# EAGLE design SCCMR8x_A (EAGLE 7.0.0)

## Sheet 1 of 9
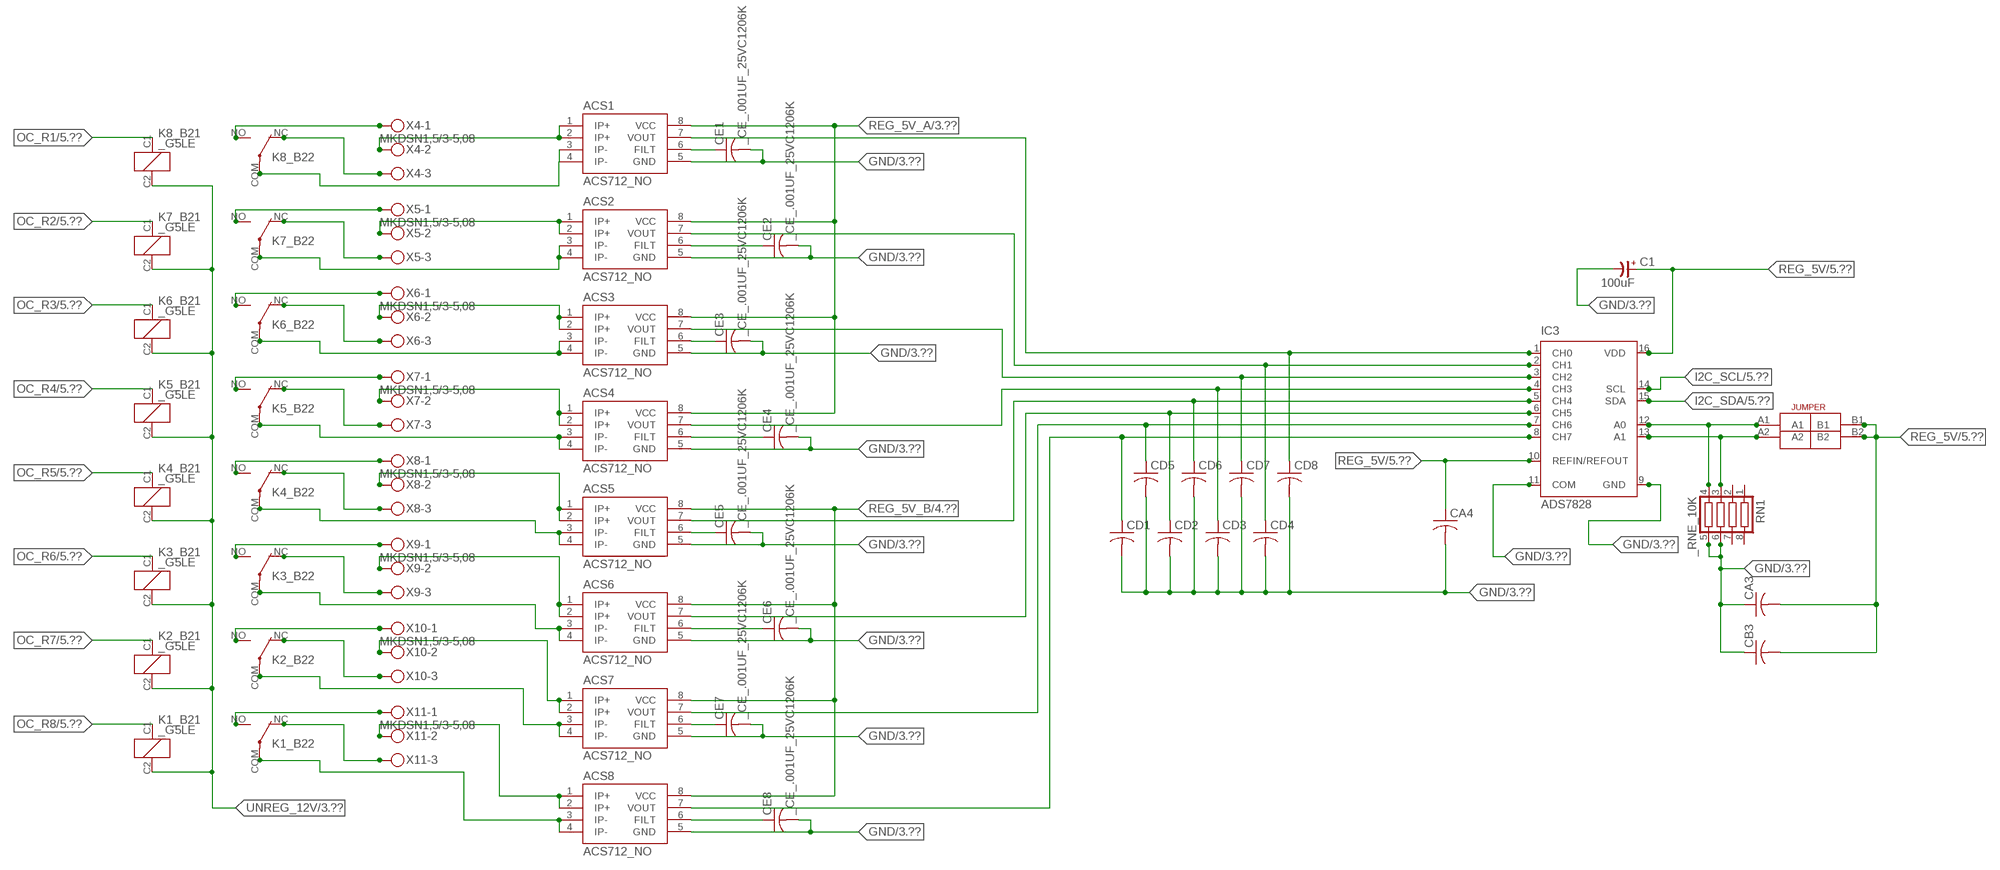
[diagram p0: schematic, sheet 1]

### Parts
ACS1  ACS712_NO  [_MA_DUAL_N-FET]
ACS2  ACS712_NO  [_MA_DUAL_N-FET]
ACS3  ACS712_NO  [_MA_DUAL_N-FET]
ACS4  ACS712_NO  [_MA_DUAL_N-FET]
ACS5  ACS712_NO  [_MA_DUAL_N-FET]
ACS6  ACS712_NO  [_MA_DUAL_N-FET]
ACS7  ACS712_NO  [_MA_DUAL_N-FET]
ACS8  ACS712_NO  [_MA_DUAL_N-FET]
C1  100uF  CP-E-025X060  [E-025X060]
CA3  CC1206KRX7R9BB104C1206K  [CC1206KRX7R9BB104]
CA4  CC1206KRX7R9BB104C1206K  [CC1206KRX7R9BB104]
CB3  TMK316F106ZL-TC1206K  [TMK316F106ZL-T]
CD1  _CD_10NF_50VC1206K  [_CD_10NF_50V]
CD2  _CD_10NF_50VC1206K  [_CD_10NF_50V]
CD3  _CD_10NF_50VC1206K  [_CD_10NF_50V]
CD4  _CD_10NF_50VC1206K  [_CD_10NF_50V]
CD5  _CD_10NF_50VC1206K  [_CD_10NF_50V]
CD6  _CD_10NF_50VC1206K  [_CD_10NF_50V]
CD7  _CD_10NF_50VC1206K  [_CD_10NF_50V]
CD8  _CD_10NF_50VC1206K  [_CD_10NF_50V]
CE1  _CE_.001UF_25VC1206K  [CE]
CE2  _CE_.001UF_25VC1206K  [CE]
CE3  _CE_.001UF_25VC1206K  [CE]
CE4  _CE_.001UF_25VC1206K  [CE]
CE5  _CE_.001UF_25VC1206K  [CE]
CE6  _CE_.001UF_25VC1206K  [CE]
CE7  _CE_.001UF_25VC1206K  [CE]
CE8  _CE_.001UF_25VC1206K  [CE]
IC3  ADS7828  [TSSOP16-PW]
K1_B2  _G5LE  [G5LE]
K2_B2  _G5LE  [G5LE]
K3_B2  _G5LE  [G5LE]
K4_B2  _G5LE  [G5LE]
K5_B2  _G5LE  [G5LE]
K6_B2  _G5LE  [G5LE]
K7_B2  _G5LE  [G5LE]
K8_B2  _G5LE  [G5LE]
RN1  _RNE_10K  [RNE]
U$4  JUMPER_2X2  [JUMPER_2X2]
X4  MKDSN1,5/3-5,08  [MKDSN1,5/3-5,08]
X5  MKDSN1,5/3-5,08  [MKDSN1,5/3-5,08]
X6  MKDSN1,5/3-5,08  [MKDSN1,5/3-5,08]
X7  MKDSN1,5/3-5,08  [MKDSN1,5/3-5,08]
X8  MKDSN1,5/3-5,08  [MKDSN1,5/3-5,08]
X9  MKDSN1,5/3-5,08  [MKDSN1,5/3-5,08]
X10  MKDSN1,5/3-5,08  [MKDSN1,5/3-5,08]
X11  MKDSN1,5/3-5,08  [MKDSN1,5/3-5,08]

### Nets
GND: ACS1.5(GND) ACS2.5(GND) ACS3.5(GND) ACS4.5(GND) ACS5.5(GND) ACS6.5(GND) ACS7.5(GND) ACS8.5(GND) C1.- CA3.1 CA4.2 CB3.1 CD1.2 CD2.2 CD3.2 CD4.2 CD5.2 CD6.2 CD7.2 CD8.2 CE1.2 CE2.2 CE3.2 CE4.2 CE5.2 CE6.2 CE7.2 CE8.2 IC3.9(GND) IC3.11(COM) RN1.5 RN1.6 ; also sheet 3,4,5,7,9
I2C_SCL: IC3.14(SCL) ; also sheet 5,7
I2C_SDA: IC3.15(SDA) ; also sheet 5,7
N$6: ACS5.7(VOUT) CD6.1 IC3.5(CH4)
N$7: ACS1.1(IP+) ACS1.2(IP+) X4.2
N$9: ACS1.7(VOUT) CD8.1 IC3.1(CH0)
N$10: ACS2.7(VOUT) CD4.1 IC3.2(CH1)
N$11: ACS3.7(VOUT) CD7.1 IC3.3(CH2)
N$12: ACS4.7(VOUT) CD3.1 IC3.4(CH3)
N$13: ACS2.1(IP+) ACS2.2(IP+) X5.2
N$14: ACS6.7(VOUT) CD2.1 IC3.6(CH5)
N$15: ACS7.7(VOUT) CD5.1 IC3.7(CH6)
N$17: IC3.12(A0) RN1.4 U$4.A1
N$18: IC3.13(A1) RN1.3 U$4.A2
N$21: ACS4.1(IP+) ACS4.2(IP+) X7.2
N$22: ACS4.3(IP-) ACS4.4(IP-) K5_B2.COM(2:COM)
N$23: ACS5.1(IP+) ACS5.2(IP+) X8.2
N$24: ACS7.1(IP+) ACS7.2(IP+) X10.2
N$25: ACS6.1(IP+) ACS6.2(IP+) X9.2
N$29: ACS8.1(IP+) ACS8.2(IP+) X11.2
N$33: ACS1.6(FILT) CE1.1
N$34: ACS2.6(FILT) CE2.1
N$35: ACS3.6(FILT) CE3.1
N$36: ACS4.6(FILT) CE4.1
N$37: ACS8.7(VOUT) CD1.1 IC3.8(CH7)
N$38: ACS5.6(FILT) CE5.1
N$39: ACS6.6(FILT) CE6.1
N$40: ACS7.6(FILT) CE7.1
N$41: ACS8.6(FILT) CE8.1
N$42: ACS1.3(IP-) ACS1.4(IP-) K8_B2.COM(2:COM)
N$43: K8_B2.NC(2:NC) X4.3
N$44: K8_B2.NO(2:NO) X4.1
N$45: K7_B2.NO(2:NO) X5.1
N$46: K6_B2.NO(2:NO) X6.1
N$137: K7_B2.NC(2:NC) X5.3
N$138: ACS2.3(IP-) ACS2.4(IP-) K7_B2.COM(2:COM)
N$139: K6_B2.NC(2:NC) X6.3
N$140: ACS3.3(IP-) ACS3.4(IP-) K6_B2.COM(2:COM)
N$141: K5_B2.NC(2:NC) X7.3
N$143: K5_B2.NO(2:NO) X7.1
N$144: K4_B2.NO(2:NO) X8.1
N$145: K4_B2.NC(2:NC) X8.3
N$146: ACS5.3(IP-) ACS5.4(IP-) K4_B2.COM(2:COM)
N$147: K3_B2.NO(2:NO) X9.1
N$148: K3_B2.NC(2:NC) X9.3
N$149: ACS6.3(IP-) ACS6.4(IP-) K3_B2.COM(2:COM)
N$150: K2_B2.NO(2:NO) X10.1
N$151: K2_B2.NC(2:NC) X10.3
N$152: ACS7.3(IP-) ACS7.4(IP-) K2_B2.COM(2:COM)
N$153: K1_B2.NO(2:NO) X11.1
N$154: K1_B2.NC(2:NC) X11.3
N$155: ACS8.3(IP-) ACS8.4(IP-) K1_B2.COM(2:COM)
N$166: ACS3.1(IP+) ACS3.2(IP+) X6.2
OC_R1: K8_B2.C1(1:C1) ; also sheet 5
OC_R2: K7_B2.C1(1:C1) ; also sheet 5
OC_R3: K6_B2.C1(1:C1) ; also sheet 5
OC_R4: K5_B2.C1(1:C1) ; also sheet 5
OC_R5: K4_B2.C1(1:C1) ; also sheet 5
OC_R6: K3_B2.C1(1:C1) ; also sheet 5
OC_R7: K2_B2.C1(1:C1) ; also sheet 5
OC_R8: K1_B2.C1(1:C1) ; also sheet 5
REG_5V: C1.+ CA3.2 CA4.1 CB3.2 IC3.10(REFIN/REFOUT) IC3.16(VDD) U$4.B1 U$4.B2 ; also sheet 5,7,9
REG_5V_A: ACS1.8(VCC) ACS2.8(VCC) ACS3.8(VCC) ACS4.8(VCC) ; also sheet 3
REG_5V_B: ACS5.8(VCC) ACS6.8(VCC) ACS7.8(VCC) ACS8.8(VCC) ; also sheet 4
UNREG_12V: K1_B2.C2(1:C2) K2_B2.C2(1:C2) K3_B2.C2(1:C2) K4_B2.C2(1:C2) K5_B2.C2(1:C2) K6_B2.C2(1:C2) K7_B2.C2(1:C2) K8_B2.C2(1:C2) ; also sheet 3,4,5,7
Unconnected: RN1.1 RN1.2 RN1.7 RN1.8

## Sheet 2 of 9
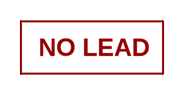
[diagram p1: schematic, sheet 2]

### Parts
U$16  NOPB_LOGO_SYM  [NOPB_LOGO_SYM]

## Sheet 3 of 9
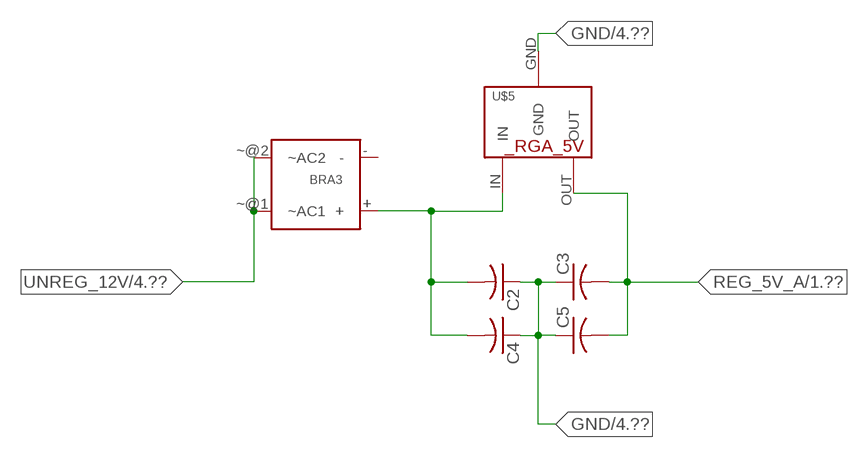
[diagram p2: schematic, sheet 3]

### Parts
BRA3  MB2S_  [MB2S]
C2  _CA_.10UF_50VC1206K  [_CA_.1UF_50V]
C3  _CA_.10UF_50VC1206K  [_CA_.1UF_50V]
C4  _CB_10UF_25VC1206K  [_CB_10UF_25V]
C5  _CB_10UF_25VC1206K  [_CB_10UF_25V]
U$5  _RGA_5V  [_RGA_5V]

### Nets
GND: C2.1 C3.1 C4.1 C5.1 U$5.GND ; also sheet 1,4,5,7,9
N$31: BRA3.+ C2.2 C4.2 U$5.IN
REG_5V_A: C3.2 C5.2 U$5.OUT ; also sheet 1
UNREG_12V: BRA3.~@1(~AC1) BRA3.~@2(~AC2) ; also sheet 1,4,5,7
Unconnected: BRA3.-

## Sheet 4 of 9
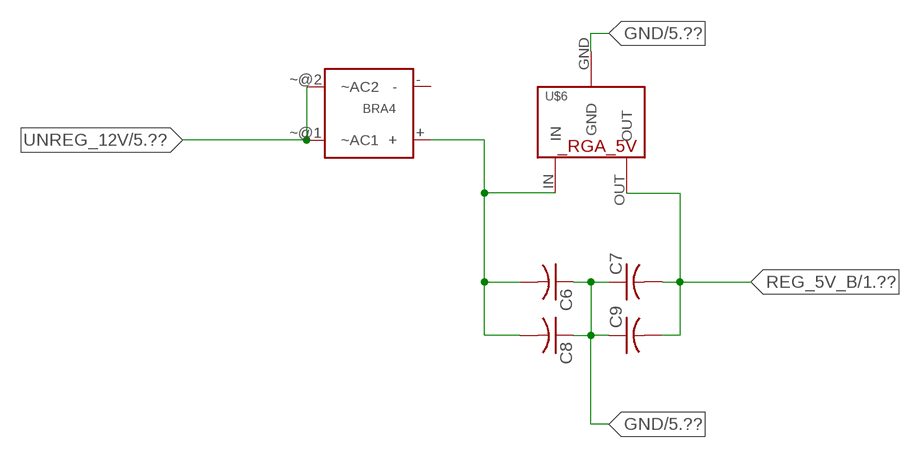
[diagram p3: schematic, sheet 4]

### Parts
BRA4  MB2S_  [MB2S]
C6  _CA_.10UF_50VC1206K  [_CA_.1UF_50V]
C7  _CA_.10UF_50VC1206K  [_CA_.1UF_50V]
C8  _CB_10UF_25VC1206K  [_CB_10UF_25V]
C9  _CB_10UF_25VC1206K  [_CB_10UF_25V]
U$6  _RGA_5V  [_RGA_5V]

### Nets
GND: C6.1 C7.1 C8.1 C9.1 U$6.GND ; also sheet 1,3,5,7,9
N$32: BRA4.+ C6.2 C8.2 U$6.IN
REG_5V_B: C7.2 C9.2 U$6.OUT ; also sheet 1
UNREG_12V: BRA4.~@1(~AC1) BRA4.~@2(~AC2) ; also sheet 1,3,5,7
Unconnected: BRA4.-

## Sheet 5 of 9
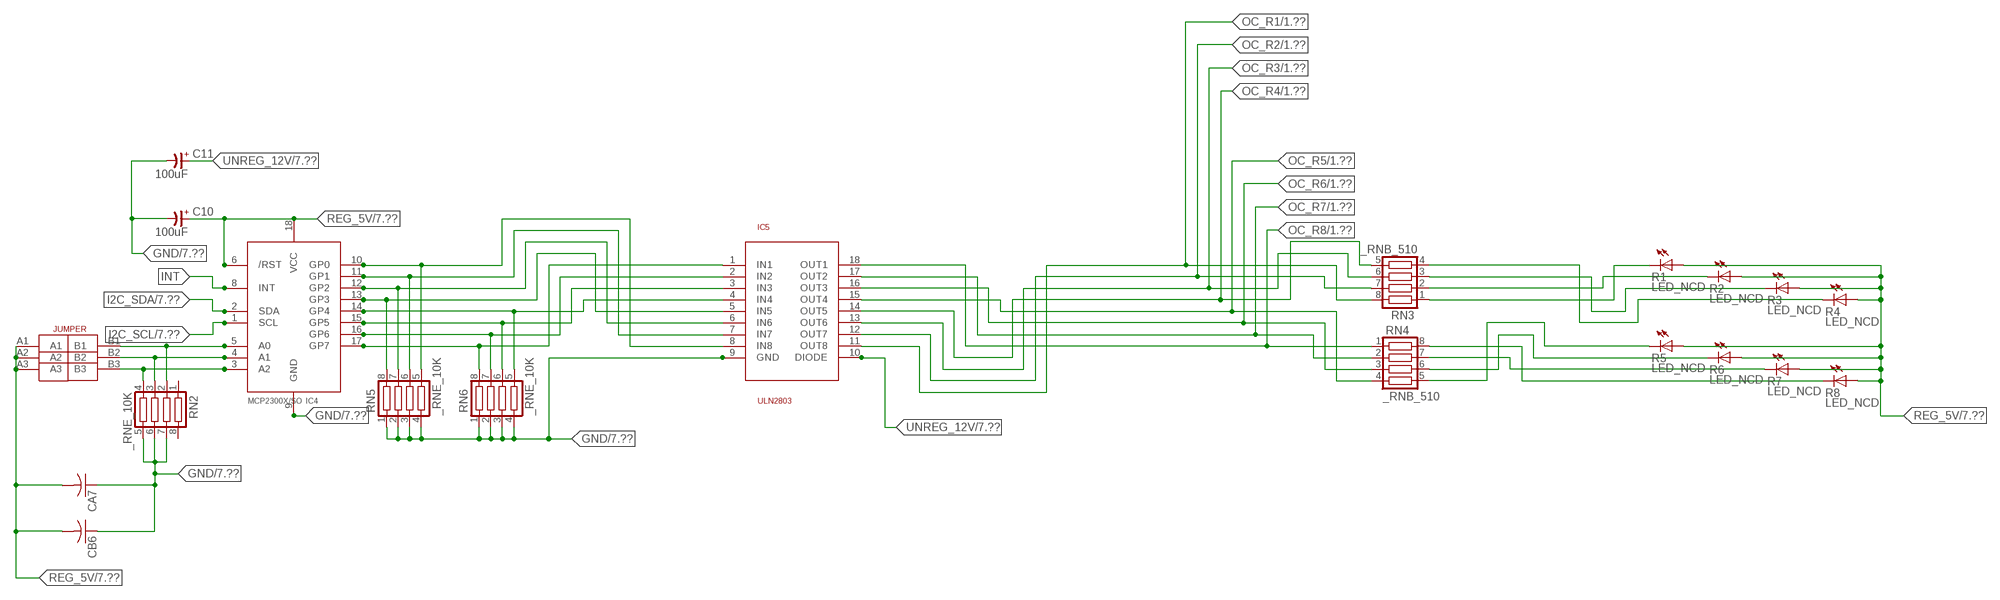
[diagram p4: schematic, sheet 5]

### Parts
C10  100uF  CP-E-025X060  [E-025X060]
C11  100uF  CP-E-025X060  [E-025X060]
CA7  CC1206KRX7R9BB104C1206K  [CC1206KRX7R9BB104]
CB6  TMK316F106ZL-TC1206K  [TMK316F106ZL-T]
IC4  MCP2300X/SO  [SO18W]
IC5  ULN2803  [SO18L]
R1  LED_NCD  [CHIPLED_0603]
R2  LED_NCD  [CHIPLED_0603]
R3  LED_NCD  [CHIPLED_0603]
R4  LED_NCD  [CHIPLED_0603]
R5  LED_NCD  [CHIPLED_0603]
R6  LED_NCD  [CHIPLED_0603]
R7  LED_NCD  [CHIPLED_0603]
R8  LED_NCD  [CHIPLED_0603]
RN2  _RNE_10K  [RNE]
RN3  _RNB_510  [RNB]
RN4  _RNB_510  [RNB]
RN5  _RNE_10K  [RNE]
RN6  _RNE_10K  [RNE]
U$18  JUMPER_3X2  [JUMPER_3X2]

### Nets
GND: C10.- C11.- CA7.1 CB6.1 IC4.9(GND) IC5.9(GND) RN2.5 RN2.6 RN2.7 RN5.1 RN5.2 RN5.3 RN5.4 RN6.1 RN6.2 RN6.3 RN6.4 ; also sheet 1,3,4,7,9
GP4: IC4.14(GP4) IC5.4(IN4) RN6.5
GP6: IC4.16(GP6) IC5.2(IN2) RN6.7
I2C_SCL: IC4.1(SCL) ; also sheet 1,7
I2C_SDA: IC4.2(SDA) ; also sheet 1,7
INT: IC4.8(INT)
N$47: IC4.5(A0) RN2.2 U$18.B1
N$48: IC4.4(A1) RN2.3 U$18.B2
N$49: IC4.3(A2) RN2.4 U$18.B3
N$50: IC4.12(GP2) IC5.6(IN6) RN5.7
N$51: IC4.11(GP1) IC5.7(IN7) RN5.6
N$52: IC4.10(GP0) IC5.8(IN8) RN5.5
N$53: R1.C RN3.1
N$54: R2.C RN3.2
N$55: R3.C RN3.3
N$56: R4.C RN3.4
N$57: R8.C RN4.8
N$81: R7.C RN4.7
N$82: R6.C RN4.6
N$83: R5.C RN4.5
N$89: IC4.13(GP3) IC5.5(IN5) RN5.8
N$93: IC4.15(GP5) IC5.3(IN3) RN6.6
N$94: IC4.17(GP7) IC5.1(IN1) RN6.8
OC_R1: IC5.11(OUT8) RN3.8 ; also sheet 1
OC_R2: IC5.12(OUT7) RN3.7 ; also sheet 1
OC_R3: IC5.13(OUT6) RN3.6 ; also sheet 1
OC_R4: IC5.14(OUT5) RN3.5 ; also sheet 1
OC_R5: IC5.15(OUT4) RN4.4 ; also sheet 1
OC_R6: IC5.16(OUT3) RN4.3 ; also sheet 1
OC_R7: IC5.17(OUT2) RN4.2 ; also sheet 1
OC_R8: IC5.18(OUT1) RN4.1 ; also sheet 1
REG_5V: C10.+ CA7.2 CB6.2 IC4.6(/RST) IC4.18(VCC) R1.A R2.A R3.A R4.A R5.A R6.A R7.A R8.A U$18.A1 U$18.A2 U$18.A3 ; also sheet 1,7,9
UNREG_12V: C11.+ IC5.10(DIODE) ; also sheet 1,3,4,7
Unconnected: RN2.1 RN2.8

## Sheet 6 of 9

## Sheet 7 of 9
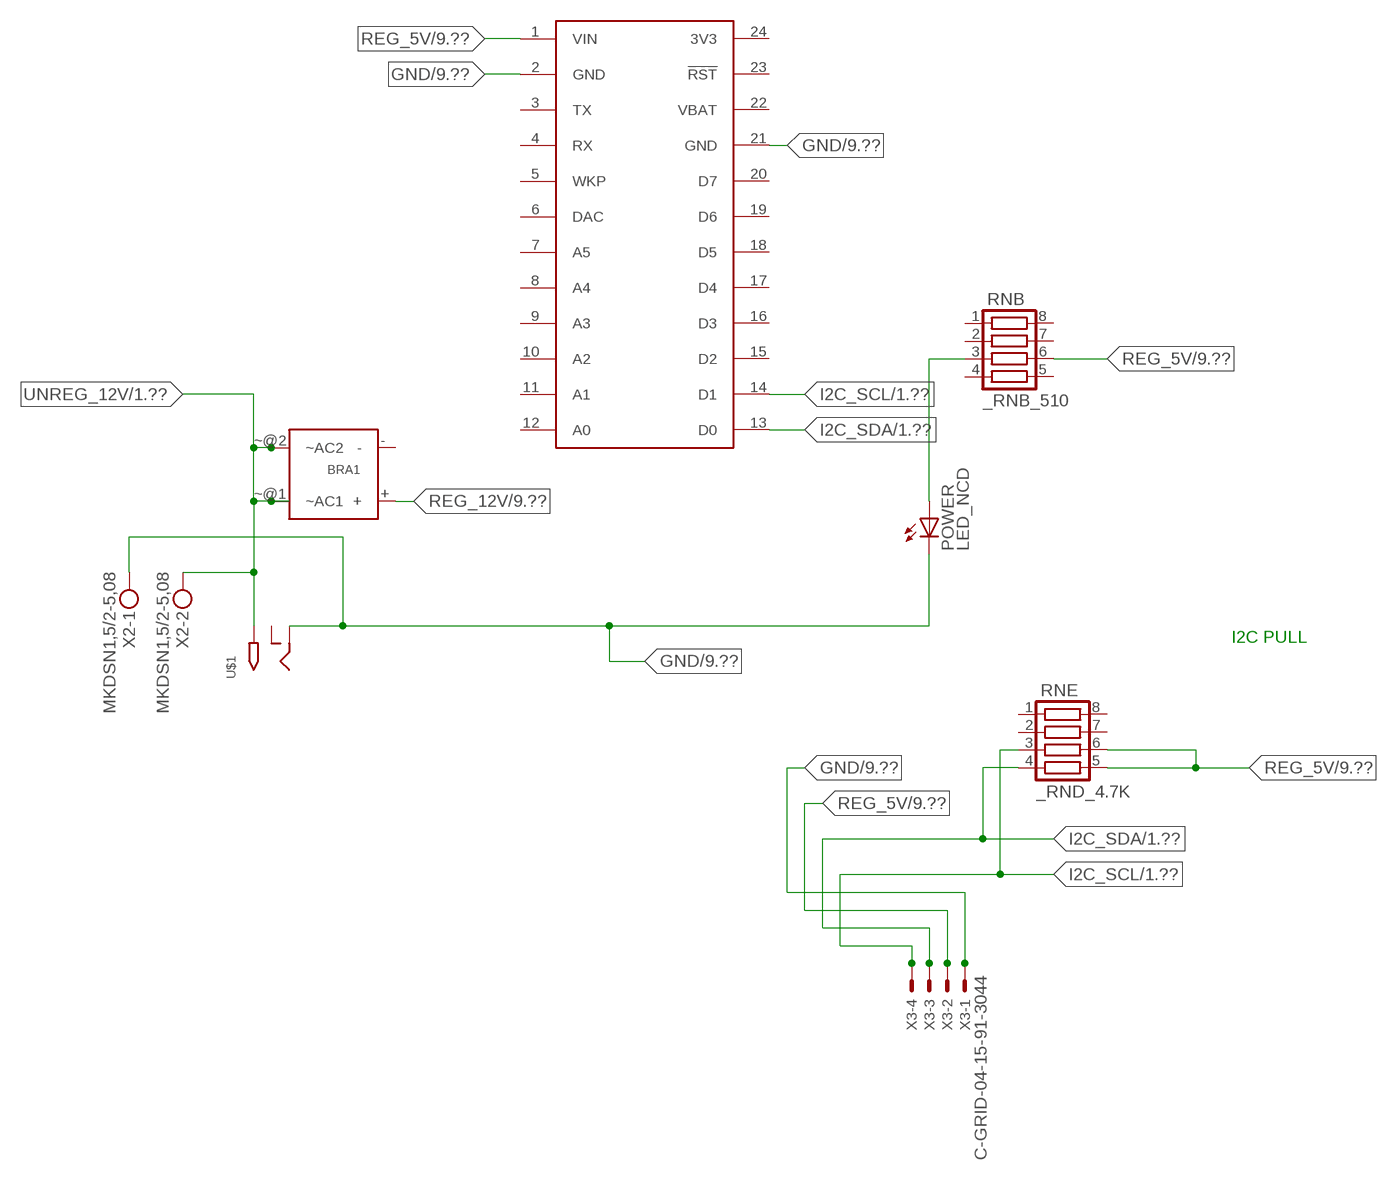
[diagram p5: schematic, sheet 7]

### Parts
BRA1  MB2S_  [MB2S]
POWER  LED_NCD  [CHIPLED_0603]
RNB  _RNB_510  [RNB]
RNE  _RND_4.7K  [RND]
S1  SPARK_CORECORE  [SPARK_CORE]
U$1  2.1MMJACK  [PJ-102A]
X2  MKDSN1,5/2-5,08  [MKDSN1,5/2-5,08]
X3  C-GRID-04-15-91-3044  [15-91-04]

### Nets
GND: POWER.C S1.2(GND) S1.21(GND) U$1.RING X2.1 X3.1 ; also sheet 1,3,4,5,9
I2C_SCL: RNE.3 S1.14(D1) X3.4 ; also sheet 1,5
I2C_SDA: RNE.4 S1.13(D0) X3.3 ; also sheet 1,5
N$2: POWER.A RNB.3
REG_5V: RNB.6 RNE.5 RNE.6 S1.1(VIN) X3.2 ; also sheet 1,5,9
REG_12V: BRA1.+ ; also sheet 9
UNREG_12V: BRA1.~@1(~AC1) BRA1.~@2(~AC2) U$1.TIP X2.2 ; also sheet 1,3,4,5
Unconnected: BRA1.- RNB.1 RNB.2 RNB.4 RNB.5 RNB.7 RNB.8 RNE.1 RNE.2 RNE.7 RNE.8 S1.3(TX) S1.4(RX) S1.5(WKP) S1.6(DAC) S1.7(A5) S1.8(A4) S1.9(A3) S1.10(A2) S1.11(A1) S1.12(A0) S1.15(D2) S1.16(D3) S1.17(D4) S1.18(D5) S1.19(D6) S1.20(D7) S1.23(!RST) U$1.RING_SW

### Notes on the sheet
- I2C PULL

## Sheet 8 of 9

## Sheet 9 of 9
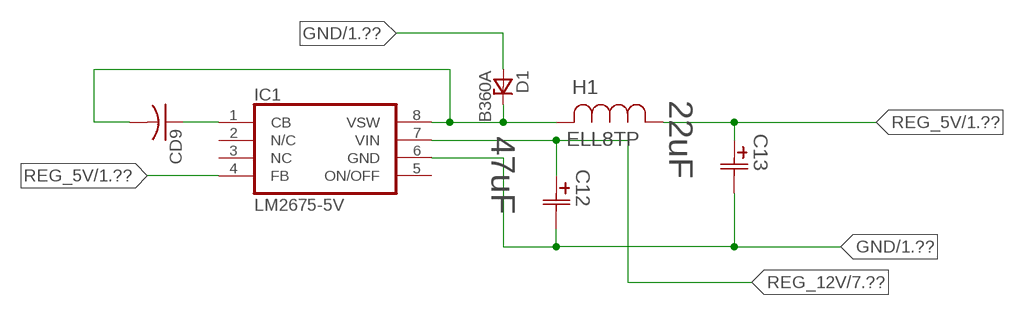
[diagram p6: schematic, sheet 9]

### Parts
C12  47uF  490-5463-6-NDCAP  [C2917(7343)-Y]
C13  22uF  490-5463-6-NDCAP  [C2917(7343)-Y]
CD9  _CD_10NF_50VC1206K  [_CD_10NF_50V]
D1  B360A  [DO214AC_ZENER]
H1  ELL8TP  [IND_ELL8TP]
IC1  LM2675-5V  LM2675  [SO-8]

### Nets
GND: C12.2(C2) C13.2(C2) D1.A IC1.6(GND) ; also sheet 1,3,4,5,7
N$1: CD9.2 D1.C H1.2 IC1.8(VSW)
N$3: CD9.1 IC1.1(CB)
REG_5V: C13.1(C1) H1.1 IC1.4(FB) ; also sheet 1,5,7
REG_12V: C12.1(C1) IC1.7(VIN) ; also sheet 7
Unconnected: IC1.2(N/C) IC1.5(ON/OFF)

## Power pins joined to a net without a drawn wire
3V3: S1.24(3V3)
NC: IC1.3(NC)
VBAT: S1.22(VBAT)

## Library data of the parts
ACS1-ACS8 = NCD_ULTIMATE_LIBRARY:ACS712_NO: Semiconductor Sensor Current Hall-effect-based isolated linear current sensor Digikey 620-1190-2-ND/ACS712ELCTR-20A-T
BRA1 BRA3 BRA4 = NCD_ULTIMATE_LIBRARY:MB2S: Bridge Rectifier BRA MB2S 200V 500ma Digikey MB2S-TPMSTR-ND/MB2S-TP
C1 C10 C11 = NCD_ULTIMATE_LIBRARY:CP-: Capacitors All Kinds POLARIZED CAP
C2 C3 C6 C7 = NCD_ULTIMATE_LIBRARY:_CA_.10UF_50V: Capacitor .1uF SMT
C4 C5 C8 C9 = NCD_ULTIMATE_LIBRARY:_CB_10UF_25V: Capacitor 10uF SMT
C12 C13 = NCD_ULTIMATE_bhaskar:490-5463-6-ND: NCD CAP
CA3 CA4 CA7 = NCD_ULTIMATE_LIBRARY:CC1206KRX7R9BB104: Capacitor CA .1uF 50V SMT C1206K CC1206KRX7R9BB104
CB3 CB6 = NCD_ULTIMATE_LIBRARY:TMK316F106ZL-T: Capacitor CB 10uF SMT 1206 TMK316F106ZL-T
CD1-CD9 = NCD_ULTIMATE_LIBRARY:_CD_10NF_50V: Capacitor 10nF SMT
CE1-CE8 = NCD_ULTIMATE_LIBRARY:_CE_.001UF_25V: Capacitor .001uF SMT
D1 = NCD_ULTIMATE_bhaskar:B360A: NCD DIODE B350A/B360A
H1 = NCD_ULTIMATE_bhaskar:ELL8TP: NCD coil
IC1 = NCD_ULTIMATE_bhaskar:LM2675: LM2675 NCD http://www.ti.com/lit/ds/symlink/lm2675.pdf
IC3 = NCD_ULTIMATE_LIBRARY:ADS7828: Semiconductor ADC I2C 12-Bit, 8-Channel Sampling ANALOG-TO-DIGITAL CONVERTER Digikey 296-12402-2-ND Source: www.ti.com .. ADS7828.pdf / ADS7828E/250; MF: TEXAS INSTRUMENTS; MPN: ADS7828E/250; OC_FARNELL: 1470338; OC_NEWARK: 74C7158
IC4 = NCD_ULTIMATE_LIBRARY:MCP2300X: Semiconductor Port Expander I/O 8-Bit I2C MCP23008 Inexpensive i2c i/o expander - 8 general purpose i/o pins with optional pullups
IC5 = NCD_ULTIMATE_LIBRARY:ULN2803: Semiconductor 8 O.C. N-Channel Transistor Driver Digikey ULN2803AFWGCELTR-ND/ULN2803AFWG,C,EL
K1_B2 K2_B2 K3_B2 K4_B2 K5_B2 K6_B2 K7_B2 K8_B2 = NCD_ULTIMATE_LIBRARY:_G5LE: Relay 5A/10A SPDT; OC_FARNELL: unknown; OC_NEWARK: unknown
POWER = NCD_ULTIMATE_bhaskar:LED_NCD
R1-R8 = NCD_ULTIMATE_LIBRARY:LED_NCD: LED Digikey 754-1132-2-ND/APT2012SRCPRV
RN1 RN2 RN5 RN6 = NCD_ULTIMATE_LIBRARY:_RNE_10K: Resistor Array RNE SMT 10K x 4 Single Resistor Source: http://www.ctscorp.com/components/Datasheets/CTSChipArrayDs.pdf Digikey 742C083103JPTR-ND/742C083103JP; OC_FARNELL: unknown; OC_NEWARK: unknown
RN3 RN4 RNB = NCD_ULTIMATE_LIBRARY:_RNB_510: Resistor Array RNB SMT 510 x 4 Single Resistor Source: http://www.ctscorp.com/components/Datasheets/CTSChipArrayDs.pdf Digikey 742C083511JPTR-ND/ 742C083511JP; OC_FARNELL: unknown; OC_NEWARK: unknown
RNE = NCD_ULTIMATE_LIBRARY:_RND_4.7K: Resistor Array RND SMT 4.7K x 4 Single Resistor Source: http://www.ctscorp.com/components/Datasheets/CTSChipArrayDs.pdf Digikey 742C083472JPTR-ND/742C083472JP; OC_FARNELL: unknown; OC_NEWARK: unknown
S1 = Spark:SPARK_CORE
U$1 = NCD_ULTIMATE_CONNECTORS:2.1MMJACK: 2.1mm x 5.5mm DC jack with internal switch. Digikey part #PJ-102A, 4UCON part #05537 By microbuilder.eu
U$4 = NCD_ULTIMATE_CONNECTORS:JUMPER_2X2
U$5 U$6 = NCD_ULTIMATE_LIBRARY:_RGA_5V: Regulator Linear 5V Digikey 497-7255-2-ND/ L7805CDT-TR
U$16 = PatternAgents-Logos:NOPB_LOGO_SYM: NOPB_LOGO_SYM
U$18 = NCD_ULTIMATE_CONNECTORS:JUMPER_3X2
X2 = NCD_ULTIMATE_CONNECTORS:MKDSN1,5/2-5,08: MKDSN 1,5/ 2-5,08 Printklemme
X3 = NCD_ULTIMATE_CONNECTORS:C-GRID-04: CONNECTOR 4-Pos I2C wire to board 2.54 mm (0.100") pitch header Digikey WM1342-ND/0015912045; OC_FARNELL: unknown; OC_NEWARK: unknown
X4-X11 = NCD_ULTIMATE_CONNECTORS:MKDSN1,5/3-5,08: MKDSN 1,5/ 3-5,08 Printklemme Nennstrom: 13,5 A Nennspannung: 250 V Rastermaß: 5,08 mm Polzahl: 3 Anschlussart: Schraubanschluss Montage: Löten Anschlussrichtung Leiter/Platine: 0 ° Artikelnummer: 1729131 Source: http://eshop.phoenixcontact.com .. 1729131.pdf

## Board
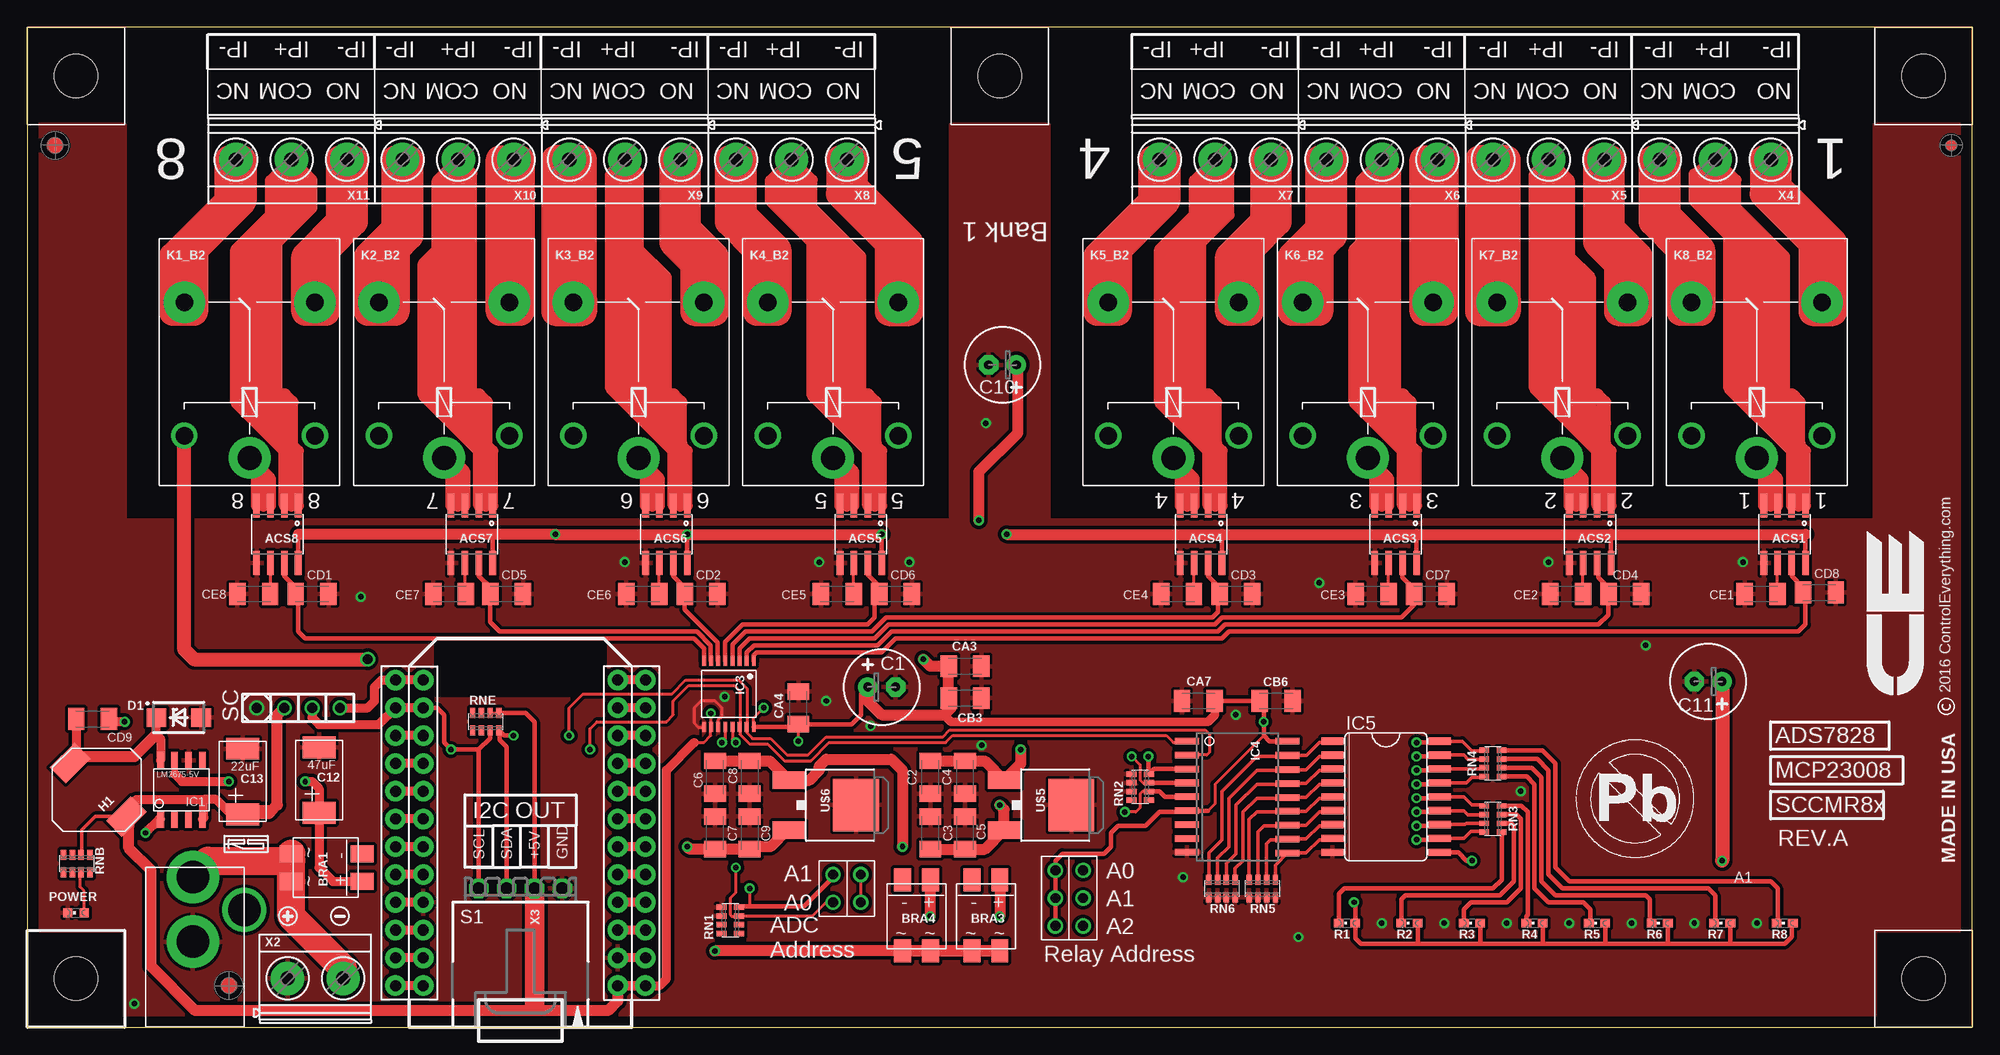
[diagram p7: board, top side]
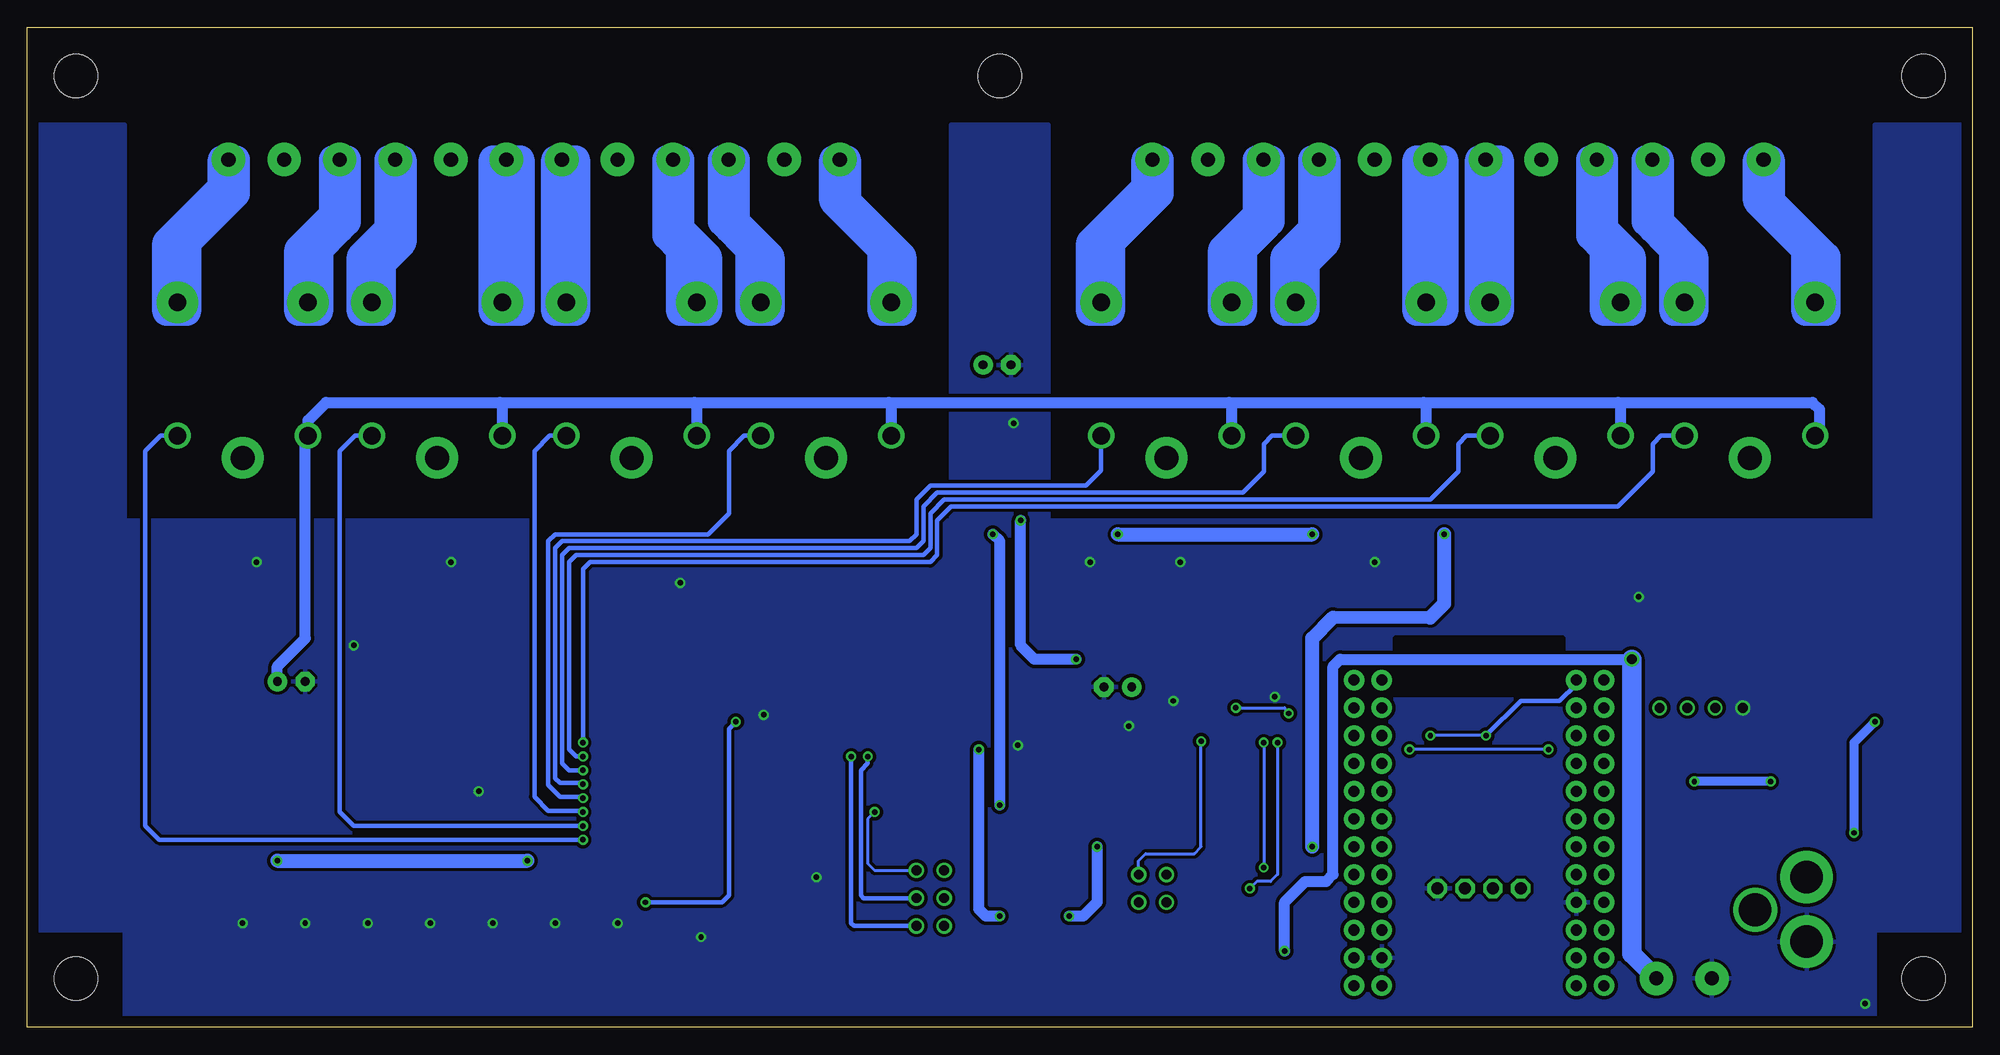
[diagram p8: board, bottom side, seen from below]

Size 177.8 x 91.44 mm. Coordinates in mm from the lower left corner, seen from the top.
Outline: 0,91.11 0,90.17
Outline: 0,90.17 0,0 177.8,0 177.8,91.44 0,91.44 0,90.17
Copper layers (1*16): Top 0.035mm / dielectric 1.5mm / Bottom 0.035mm
Design rules "default": minimum track width 10mil, minimum drill 24mil, track to track 8mil, track to pad 8mil, pad to pad 8mil, via to via 8mil, smd to smd 8mil, copper to edge 40mil, drill to drill 8mil, minimum pad ring 10mil, minimum via ring 8mil, stop-mask expansion 4mil, vias tented up to drill 0mil, thermal gap 10mil
Holes 3.96 mm at 4.45,4.45 4.45,4.45

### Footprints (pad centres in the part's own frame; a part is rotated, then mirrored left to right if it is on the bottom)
_MA_DUAL_N-FET = smd 0.61 x 2.21: 1 -1.905,-2.616; 2 -0.635,-2.616; 3 0.635,-2.616; 4 1.905,-2.616; 5 1.905,2.616; 6 0.635,2.616; 7 -0.635,2.616; 8 -1.905,2.616
MB2S = smd 1.55 x 2.1: + 0,-6.5; - 2.54,-6.5; ~@1 0,0; ~@2 2.54,0
E-025X060 = drill 0.813 pad 1.778: + -1.27,0 | drill 0.813 pad 1.778 octagon: - 1.27,0
_CA_.1UF_50V = smd 1.5 x 2: 1 -1.5,0; 2 1.5,0
_CB_10UF_25V = smd 1.5 x 2: 1 -1.5,0; 2 1.5,0
C2917(7343)-Y = smd 2 x 3: 1 -3,0; 2 3,0
CC1206KRX7R9BB104 = smd 1.5 x 2: 1 -1.5,0; 2 1.5,0
TMK316F106ZL-T = smd 1.5 x 2: 1 -1.5,0; 2 1.5,0
_CD_10NF_50V = smd 1.5 x 2: 1 -1.5,0; 2 1.5,0
CE = smd 1.5 x 2: 1 -1.5,0; 2 1.5,0
DO214AC_ZENER = smd 1.8 x 1.7: A 2.05,0; C -2.05,0
IND_ELL8TP = smd 2.054 x 3.2 rotated 45: 1 -2.442,-2.696; 2 2.442,2.442
SO-8 = smd 0.6 x 1.55: 1 -1.905,-2.69; 2 -0.635,-2.69; 3 0.635,-2.69; 4 1.905,-2.69; 5 1.905,2.71; 6 0.635,2.71; 7 -0.635,2.71; 8 -1.905,2.71
TSSOP16-PW = smd 0.35 x 0.9: 1 -2.275,-3.025; 2 -1.625,-3.025; 3 -0.975,-3.025; 4 -0.325,-3.025; 5 0.325,-3.025; 6 0.975,-3.025; 7 1.625,-3.025; 8 2.275,-3.025; 9 2.275,3.025; 10 1.625,3.025; 11 0.975,3.025; 12 0.325,3.025; 13 -0.325,3.025; 14 -0.975,3.025; 15 -1.625,3.025; 16 -2.275,3.025
SO18W = smd 0.6 x 2.2: 1 -4.445,-4.6; 2 -3.175,-4.6; 3 -1.905,-4.6; 4 -0.635,-4.6; 5 0.635,-4.6; 6 1.905,-4.6; 7 3.175,-4.6; 8 4.445,-4.6; 9 5.715,-4.6; 10 5.775,4.6; 11 4.505,4.6; 12 3.235,4.6; 13 1.965,4.6; 14 0.695,4.6; 15 -0.575,4.6; 16 -1.845,4.6; 17 -3.145,4.6; 18 -4.445,4.6
SO18L = smd 0.66 x 2.032: 1 -5.08,-4.902; 2 -3.81,-4.902; 3 -2.54,-4.902; 4 -1.27,-4.902; 5 0,-4.902; 6 1.27,-4.902; 7 2.54,-4.902; 8 3.81,-4.902; 9 5.08,-4.902; 10 5.08,4.902; 11 3.81,4.902; 12 2.54,4.902; 13 1.27,4.902; 14 0,4.902; 15 -1.27,4.902; 16 -2.54,4.902; 17 -3.81,4.902; 18 -5.08,4.902
G5LE = drill 1.6: C1 -7.493,-5.969; C2 -7.493,5.969 | drill 2.2 pad 3.81: COM -9.525,0 | drill 1.6 pad 3.81: NC 4.699,5.969; NO 4.699,-5.969
CHIPLED_0603 = smd 0.8 x 0.8: A 0,-0.75; C 0,0.75
CHIPLED_0603' = smd 0.8 x 0.876: A 0,-0.75; C 0,0.75
RNE = smd 0.5 x 0.9: 1 -1.2,-0.8; 2 -0.4,-0.8; 3 0.4,-0.8; 4 1.2,-0.8; 5 1.2,0.8; 6 0.4,0.8; 7 -0.4,0.8; 8 -1.2,0.8
RNB = smd 0.5 x 0.9: 1 -1.2,-0.8; 2 -0.4,-0.8; 3 0.4,-0.8; 4 1.2,-0.8; 5 1.2,0.8; 6 0.4,0.8; 7 -0.4,0.8; 8 -1.2,0.8
RND = smd 0.5 x 0.9: 1 -1.2,-0.8; 2 -0.4,-0.8; 3 0.4,-0.8; 4 1.2,-0.8; 5 1.2,0.8; 6 0.4,0.8; 7 -0.4,0.8; 8 -1.2,0.8
SPARK_CORE = drill 1.016 pad 1.88: 1 -8.89,13.97; 2 -8.89,11.43; 3 -8.89,8.89; 4 -8.89,6.35; 5 -8.89,3.81; 6 -8.89,1.27; 7 -8.89,-1.27; 8 -8.89,-3.81; 9 -8.89,-6.35; 10 -8.89,-8.89; 11 -8.89,-11.43; 12 -8.89,-13.97; 13 8.89,-13.97; 14 8.89,-11.43; 15 8.89,-8.89; 16 8.89,-6.35; 17 8.89,-3.81; 18 8.89,-1.27; 19 8.89,1.27; 20 8.89,3.81; 21 8.89,6.35; 22 8.89,8.89; 23 8.89,11.43; 24 8.89,13.97; 25 -11.43,13.97; 26 -11.43,11.43; 27 -11.43,8.89; 28 -11.43,6.35; 29 -11.43,3.81; 30 -11.43,1.27; 31 -11.43,-1.27; 32 -11.43,-3.81; 33 -11.43,-6.35; 34 -11.43,-8.89; 35 -11.43,-11.43; 36 -11.43,-13.97; 37 11.43,13.97; 38 11.43,11.43; 39 11.43,8.89; 40 11.43,6.35; 41 11.43,3.81; 42 11.43,1.27; 43 11.43,-1.27; 44 11.43,-3.81; 45 11.43,-6.35; 46 11.43,-8.89; 47 11.43,-11.43; 48 11.43,-13.97
PJ-102A = drill 3 pad 4.8: RING 0.1,-3.39; TIP 0.1,-9.29 | drill 3 pad 3.251: RING_SW -4.6,-6.29
JUMPER_2X2 = drill 0.9: A1 0,2.54; A2 0,0; B1 2.54,2.54; B2 2.54,0
_RGA_5V = smd 4.826 x 4.191: GND 0,2.096 | smd 1.6 x 3: IN -2.28,-4.04; OUT 2.28,-4.04
PCB_MOUNTING_HOLE = hole 3.962: 4.445,4.445
JUMPER_3X2 = drill 0.9: A1 0,5.08; A2 0,2.54; A3 0,0; B1 2.54,5.08; B2 2.54,2.54; B3 2.54,0
MKDSN1,5/2-5,08 = drill 1.3 pad 3.048: 1 -2.561,0.025; 2 2.519,0.025
15-91-04 = drill 1.1 pad 1.778 octagon: 1 -3.81,-7.62; 2 -1.27,-7.62; 3 1.27,-7.62; 4 3.81,-7.62
MKDSN1,5/3-5,08 = drill 1.3 pad 3.048: 1 -7.641,0.025; 2 -2.561,0.025; 3 2.519,0.025

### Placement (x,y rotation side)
ACS1  160.66,45.09 180 top
ACS2  142.88,45.09 180 top
ACS3  125.09,45.09 180 top
ACS4  107.31,45.09 180 top
ACS5  76.2,45.09 180 top
ACS6  58.42,45.09 180 top
ACS7  40.64,45.09 180 top
ACS8  22.86,45.09 180 top
BRA1  24.13,13.34 90 top
BRA3  88.9,6.99 180 top
BRA4  82.55,6.99 180 top
C1  78.11,31.12 0 top
C2  82.55,22.86 90 top
C3  82.55,17.78 270 top
C4  85.72,22.86 90 top
C5  85.72,17.78 270 top
C6  62.87,22.86 90 top
C7  62.87,17.78 270 top
C8  66.04,22.86 90 top
C9  66.04,17.78 270 top
C10  89.15,60.58 180 top
C11  153.67,31.62 180 top
C12  26.67,22.61 90 top
C13  19.68,22.48 90 top
CA3  85.72,33.02 180 top
CA4  70.48,29.21 90 top
CA7  107.06,29.84 0 top
CB3  85.72,30.1 180 top
CB6  114.17,29.84 180 top
CD1  26.04,39.62 0 top
CD2  61.59,39.62 0 top
CD3  110.49,39.62 0 top
CD4  146.05,39.62 0 top
CD5  43.81,39.62 0 top
CD6  79.38,39.62 0 top
CD7  128.27,39.62 0 top
CD8  163.83,39.75 0 top
CD9  5.97,28.19 180 top
CE1  158.5,39.62 180 top
CE2  140.72,39.62 180 top
CE3  122.94,39.62 180 top
CE4  105.16,39.62 180 top
CE5  74.04,39.62 180 top
CE6  56.26,39.62 180 top
CE7  38.61,39.62 180 top
CE8  20.7,39.62 180 top
D1  13.84,28.32 0 top
H1  6.35,21.72 90 top
IC1  14.1,21.72 0 top
IC3  64.14,30.48 180 top
IC4  110.62,21.72 270 top
IC5  124.21,21.08 270 top
K1_B2  20.32,61.59 90 top
K2_B2  38.1,61.59 90 top
K3_B2  55.88,61.59 90 top
K4_B2  73.66,61.59 90 top
K5_B2  104.78,61.59 90 top
K6_B2  122.56,61.59 90 top
K7_B2  140.34,61.59 90 top
K8_B2  158.12,61.59 90 top
POWER  4.45,10.48 90 top
R1  LED_NCD  [CHIPLED_0603']  120.65,9.53 90 top
R2  LED_NCD  [CHIPLED_0603']  126.36,9.53 90 top
R3  LED_NCD  [CHIPLED_0603']  132.08,9.53 90 top
R4  LED_NCD  [CHIPLED_0603']  137.79,9.53 90 top
R5  LED_NCD  [CHIPLED_0603']  143.51,9.53 90 top
R6  LED_NCD  [CHIPLED_0603']  149.22,9.53 90 top
R7  LED_NCD  [CHIPLED_0603']  154.94,9.53 90 top
R8  LED_NCD  [CHIPLED_0603']  160.66,9.53 90 top
RN1  64.26,9.78 90 top
RN2  101.73,21.97 90 top
RN3  133.99,19.05 90 top
RN4  133.99,24.13 270 top
RN5  112.9,12.7 0 top
RN6  109.22,12.7 0 top
RNB  4.51,14.99 0 top
RNE  41.91,27.94 0 top
S1  45.09,17.78 180 top
U$1  15.24,4.45 180 top
U$4  73.66,11.43 0 top
U$5  93.34,20.32 270 top
U$6  73.66,20.32 270 top
U$10  [VISION_REF15]  18.41,3.81 0 top
U$15  PCB_MOUNTING_HOLE  [PCB_MOUNTING_HOLE]  177.8,0 90 top
U$16  141.38,15.06 0 top
U$18  93.98,9.27 0 top
U$20  PCB_MOUNTING_HOLE  [PCB_MOUNTING_HOLE]  177.8,82.55 90 top
U$21  [ICON_USA]  175.01,26.92 270 top
U$22  [ICON_MINUS]  28.57,10.16 180 top
U$23  PCB_MOUNTING_HOLE  [PCB_MOUNTING_HOLE]  93.34,82.55 90 top
U$24  [ICON_PLUS]  23.81,10.16 90 top
U$25  PCB_MOUNTING_HOLE  [PCB_MOUNTING_HOLE]  8.89,82.55 90 top
U$26  PCB_MOUNTING_HOLE  [PCB_MOUNTING_HOLE]  177.8,82.55 90 top
U$27  [VISION_REF15]  2.54,80.65 270 top
U$28  [VISION_REF10]  175.9,80.65 270 top
X2  26.35,4.45 0 top
X3  45.09,5.08 180 top
X4  151.76,79.38 180 top
X5  136.53,79.38 180 top
X6  121.28,79.38 180 top
X7  106.05,79.38 180 top
X8  67.31,79.38 180 top
X9  52.07,79.38 180 top
X10  36.83,79.38 180 top
X11  21.59,79.38 180 top

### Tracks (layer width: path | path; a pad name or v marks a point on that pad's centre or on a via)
GND  (via drill 0.5, 0.9)
  Top 0.254: IC3.11 63.16,28.11 63.5,28.45 63.5,29.21 62.87,29.84 61.59,29.84 60.96,29.21 60.96,27.81 61.34,27.43 61.84,27.43 IC3.9
  Top 0.61: C8.1 66.04,21.59
  other vias: 156.84,42.55 73.03,29.84 139.06,42.55 118.11,40.64 105.66,13.72 146.69,9.53 116.2,8.26 152.4,9.53 158.12,9.53 140.97,9.53 135.25,9.53 129.54,9.53 123.83,9.53 110.49,28.57 77.09,27.56 30.48,39.37 54.61,42.55 72.39,42.55 147.96,34.92 136.53,21.59 87.25,25.78 87.63,55.24 80.64,42.55 9.78,2.16 20.95,29.21 63.75,30.23
  pour Top (isolate 0.305): 8.89,-1.9 8.89,8.89 -2.54,8.89 -2.54,82.55 8.89,82.55 8.89,46.35 84.45,46.35 84.45,82.55 93.34,82.55 93.34,46.35 168.91,46.35 168.91,82.55 179.07,82.55 179.71,83.19 179.71,8.89 168.91,8.89 168.91,-1.27 168.28,-1.9
  pour Bottom (isolate 0.305): 8.89,-1.9 8.89,8.89 -10.16,8.89 -10.16,82.55 8.89,82.55 8.89,46.35 84.45,46.35 84.45,82.55 93.34,82.55 93.34,46.35 168.91,46.35 168.91,82.55 179.07,82.55 179.71,83.19 179.71,8.89 168.91,8.89 168.91,-1.27 168.28,-1.9
GP4
  Top 0.305: RN6.5 110.42,14.54 111.12,15.24 111.12,19.69 112.39,20.96 115.15,20.96 IC4.14 116.91,21.02 118.11,22.23 119.18,22.23 IC5.4
GP6
  Top 0.305: RN6.7 108.82,15.47 109.86,16.51 109.86,20.96 112.39,23.5 115.15,23.5 IC4.16 116.91,23.56 118.11,24.77 119.18,24.77 IC5.2
I2C_SCL  (via drill 0.5, 0.9)
  Top 0.254: 65.15,27.5 65.15,30.73 64.64,31.24 60.45,31.24 59.05,29.84 59.05,28.57 58.42,27.94 52.07,27.94 51.44,27.3 v51.44,25.4 | 65.15,27.5 IC3.14 | 65.15,27.5 65.15,26.8 66.04,25.91 67.69,25.91 69.22,24.38 71.63,24.38 73.28,26.04 83.95,26.04 84.58,26.67 104.14,26.67 104.78,26.04 105.89,26.04 IC4.1
  Top 0.406: X3.4 41.27,25.4 | 41.27,25.4 42.29,26.42 42.29,27.12 RNE.3 | S1.14 37.47,29.21 38.1,28.57 38.1,26.04 v38.73,25.4 41.27,25.4
  Top 0.813: v26.04,29.21 26.04,28.32 26.67,27.69 32.13,27.69 33.66,29.21
  Bottom 0.254: v38.73,25.4 v51.44,25.4
I2C_SDA  (via drill 0.5, 0.9)
  Top 0.254: 65.79,27.48 65.79,30.99 65.02,31.75 60.2,31.75 58.93,30.48 50.8,30.48 49.53,29.21 v49.53,26.67 | 65.79,27.48 IC3.15 | 65.79,27.48 65.79,26.92 66.29,26.42 67.94,26.42 69.47,24.89 71.37,24.89 73.03,26.54 83.69,26.54 84.33,27.18 107.7,27.18 108.08,26.8 108.08,25.15 107.82,24.89 IC4.2
  Top 0.406: X3.3 43.81,25.65 43.18,26.29 43.18,27.07 RNE.4 43.58,26.67 v44.45,26.67
  Top 0.813: v28.57,29.21 31.11,29.21 31.75,29.84 31.75,31.12 32.38,31.75 33.66,31.75
  Bottom 0.254: v44.45,26.67 v49.53,26.67
  Bottom 0.406: S1.13 36.2,31.37 37.72,29.84 41.27,29.84 v44.45,26.67
N$1
  Top 0.813: H1.2 3.88,24.77 | D1.C 11.79,26.78 12.19,26.38 IC1.8 | CD9.2 4.47,24.79 4.45,24.77
  Top 1.016: 3.88,24.77 4.45,24.77 9.78,24.77 11.79,26.78
N$2
  Top 0.254: POWER.A 5.2,12.46 4.83,12.83 4.83,14.1 RNB.3
  Top 0.406: 4.95,14.14 RNB.3
N$3  (via drill 0.5)
  Top 0.813: IC1.1 12.04,19.03 v10.79,17.78 | v8.89,27.94 7.72,27.94 CD9.1
  Bottom 0.813: v10.79,17.78 10.79,26.04 v8.89,27.94
N$6
  Top 0.406: IC3.5 63.81,35.23 65.41,36.83 76.83,36.83 77.47,37.47 77.47,39.22 CD6.1 77.88,40.36 76.83,41.4 ACS5.7
N$7
  Top 1.016: ACS1.1 162.56,52.7 161.93,53.34 160.66,54.61 160.66,70.49 156.21,74.93 156.21,77.47 X4.2 152.4,78.06 152.4,75.56 155.57,72.39 155.57,58.42 161.29,52.7 ACS1.2
  Top 1.27: 161.93,53.34 161.93,57.15 161.29,57.79 161.29,54.61
  Top 1.778: 154.31,79.33 X4.2
N$8
  Top 1.016: 21.59,47.62 21.59,50.16
N$9
  Top 0.406: IC3.1 66.41,34.02 66.67,34.29 78.11,34.29 79.38,35.56 109.22,35.56 109.86,36.2 161.93,36.2 162.56,36.83 162.56,39.52 CD8.1 162.33,40.23 161.29,41.27 ACS1.7
N$10
  Top 0.406: IC3.2 65.76,34.26 66.42,34.92 77.72,34.92 78.99,36.2 108.84,36.2 109.47,36.83 143.64,36.83 144.53,37.72 144.53,39.6 CD4.1 144.55,40.23 143.64,41.15 143.64,42.34 ACS2.7
N$11
  Top 0.406: IC3.3 65.11,34.63 66.04,35.56 77.47,35.56 78.74,36.83 108.58,36.83 109.22,37.47 125.6,37.47 126.75,38.61 126.75,39.6 CD7.1 126.77,40.11 125.73,41.15 ACS3.7
N$12
  Top 0.406: IC3.4 64.46,35 65.66,36.2 77.22,36.2 78.49,37.47 108.33,37.47 108.84,37.97 108.84,39.47 CD3.1 108.99,40.23 107.95,41.27 ACS4.7
N$13
  Top 1.016: ACS2.2 143.51,52.7 137.79,58.42 137.79,78.06 X5.2 140.34,78.1 140.97,77.47 140.97,70.49 142.88,68.58 142.88,57.79 142.88,56.52 142.88,54.61 144.15,53.34 144.78,52.7 ACS2.1
  Top 1.27: 144.15,53.34 144.15,55.24 | 144.15,55.24 142.88,56.52 142.88,55.24 143.51,54.61 | 144.15,55.24 144.15,57.15 143.51,57.79 142.88,57.79
N$14
  Top 0.406: ACS6.7 59.05,41.27 60.33,40.01 60.33,39.85 CD2.1 60.09,38.2 63.12,35.18 63.12,33.55 IC3.6
N$15
  Top 0.406: 41.27,42.55 ACS7.7 41.27,41.27 42.29,40.26 42.29,39.65 CD5.1 42.31,37.06 43.18,36.2 61.21,36.2 62.48,34.92 62.48,33.53 IC3.7
N$16
  Top 1.016: 24.13,47.62 24.13,52.7 22.23,54.61 22.23,57.79 22.23,72.39 25.4,75.56 25.4,77.47 24.13,78.74 22.86,77.47 22.86,74.29 19.68,71.12 19.68,57.15 20.32,56.52 | 20.32,56.52 21.59,55.24 21.59,58.42 21.59,72.39 20.32,71.12 20.32,56.52 | 20.32,56.52 20.95,56.52 20.95,71.75 23.5,74.29 | 24.13,74.93 24.77,75.56 24.77,77.47 24.13,78.1 24.13,74.93 | 24.13,74.93 23.5,74.29 | 23.5,74.29 23.5,77.47
  Top 1.27: 24.13,52.7 24.13,57.15 23.5,57.79 22.23,57.79 22.23,57.15 23.5,55.88 | 23.5,55.88 23.5,54.61 | 23.5,55.88 23.5,56.52 21.59,58.42
N$17  (via drill 0.5)
  Top 0.254: IC3.12 63.81,26.34 v63.5,26.04 | v66.04,12.7 66.04,11.05
  Top 0.406: U$4.A1 73.66,13.72 70.99,11.05 66.04,11.05 65.13,11.05 RN1.4
  Bottom 0.254: v63.5,26.04 63.5,13.97 64.14,13.34 65.41,13.34 v66.04,12.7
N$18  (via drill 0.5)
  Top 0.254: IC3.13 64.46,26.34 v64.77,26.04 | v64.77,14.61 64.77,12.32 64.26,11.81 64.26,10.29 64.39,10.16 65.04,10.16 RN1.3 | U$4.A2 73.03,11.43 71.75,10.16 65.08,10.16
  Top 0.406: 65.08,10.16 RN1.3
  Bottom 0.254: v64.77,26.04 v64.77,14.61
N$20
  Top 1.016: 39.37,50.8 39.37,47.62
N$21
  Top 1.016: ACS4.2 107.95,52.7 103.5,57.15 103.5,71.12 106.68,74.29 106.68,77.42 X7.2 109.86,78.1 109.86,74.29 107.31,71.75 107.31,54.61 108.58,53.34 109.22,52.7 ACS4.1
  Top 1.27: 108.58,53.34 108.58,57.15 107.95,57.79 107.95,54.61
N$22
  Top 1.016: ACS4.4 105.41,51.44 K5_B2.COM 106.68,50.16 ACS4.3
N$23
  Top 1.016: ACS5.2 76.83,52.7 71.75,57.79 71.75,71.75 67.94,75.56 67.94,77.42 X8.2 71.75,77.47 71.75,74.93 76.2,70.49 76.2,54.61 77.47,53.34 78.11,52.7 ACS5.1 | 75.56,54.61 75.56,55.24 72.39,58.42 72.39,72.39 68.58,76.2 68.58,77.47 69.85,78.74 71.12,77.47 71.12,74.93 75.56,70.49 75.56,57.79 75.56,55.88 73.03,58.42 73.03,71.75 | 73.03,72.39 73.03,71.75 | 73.03,71.75 74.93,69.85 74.93,57.79 | 74.93,57.15 74.93,57.79 | 74.93,57.79 73.66,59.05 73.66,70.49 74.3,69.85 74.3,59.05
  Top 1.27: 77.47,53.34 77.47,57.15 76.83,57.79 75.56,57.79 76.83,56.52 76.83,54.61
N$24
  Top 1.016: 41.91,52.7 41.91,47.62 | ACS7.2 41.27,52.7 36.2,57.79 36.2,69.85 37.47,71.12 37.47,77.42 X10.2 40.64,78.1 40.64,57.79 40.64,54.61 42.55,52.7 ACS7.1
  Top 1.27: 41.91,52.7 41.91,57.15 41.27,57.79 40.64,57.79 40.64,55.88 41.27,55.24
N$25
  Top 1.016: ACS6.2 59.05,52.7 53.34,58.42 53.34,78.06 X9.2 55.88,78.1 55.88,71.12 58.42,68.58 58.42,54.61 59.69,53.34 60.33,52.7 ACS6.1 | 53.98,78.1 53.98,58.42 57.78,54.61 57.78,67.94 54.61,71.12 54.61,78.74 55.24,78.1 55.24,58.42 | 55.24,57.79 55.24,58.42 | 55.24,58.42 54.61,59.05 54.61,70.49 57.15,67.94 57.15,57.79 57.15,55.88
  Top 1.27: 59.69,53.34 59.69,57.15 59.05,57.79 57.78,57.79 | 57.15,57.79 57.78,57.79 | 57.78,57.79 59.05,56.52 59.05,54.61
N$26
  Top 1.016: 40.01,54.61 40.01,78.1 39.37,78.74 38.1,77.47 38.1,56.52 39.37,55.24 39.37,78.1 38.73,77.47 38.73,56.52 37.47,57.79 37.47,69.85 | 37.47,70.49 37.47,69.85 | 37.47,69.85 36.83,69.22 36.83,57.79
N$29
  Top 1.016: ACS8.2 23.5,52.7 19.05,57.15 19.05,71.12 22.23,74.29 22.23,77.42 X11.2 26.04,77.47 26.04,74.93 22.86,71.75 22.86,54.61 24.77,52.7 ACS8.1
N$30
  Top 1.016: 56.52,56.52 56.52,67.94 55.88,68.58
N$31  (via drill 0.5)
  Top 1.016: C2.2 C4.2 87.55,24.36 U$5.IN 90.81,24.1 v90.81,25.4 | BRA3.+ v88.9,10.16
  Bottom 1.016: v88.9,10.16 90.17,10.16 90.81,10.79 v90.81,25.4
N$32  (via drill 0.5)
  Top 1.016: C6.2 C8.2 67.86,24.36 U$6.IN 71.5,22.6 72.39,23.5 72.39,23.88 73.03,24.51 78.99,24.51 80.01,23.5 v80.01,16.51 | v82.55,10.16 BRA4.+
  Bottom 1.016: v80.01,16.51 80.01,11.43 81.28,10.16 v82.55,10.16
N$33
  Top 0.254: CE1.1 160,42.45 ACS1.6
N$34
  Top 0.254: CE2.1 142.22,42.45 ACS2.6
N$35
  Top 0.254: CE3.1 124.44,42.45 ACS3.6
N$36
  Top 0.254: CE4.1 106.66,42.45 ACS4.6
N$37
  Top 0.406: IC3.8 61.86,34.66 60.96,35.56 25.4,35.56 24.77,36.2 24.77,39.39 CD1.1 24.54,40.23 23.5,41.27 ACS8.7
N$38
  Top 0.254: CE5.1 75.54,42.45 ACS5.6
N$39
  Top 0.254: CE6.1 57.76,42.45 ACS6.6
N$40
  Top 0.254: CE7.1 40.01,39.62 ACS7.6
N$41
  Top 0.254: CE8.1 22.23,39.62 ACS8.6
N$42
  Top 1.016: ACS1.3 160.02,50.16 K8_B2.COM 158.75,51.44 ACS1.4
N$43
  Top 1.016: K8_B2.NC 152.15,70.74 149.22,73.66 149.22,79.33 X4.3
N$44
  Top 1.016: K8_B2.NO 164.08,71.5 159.38,76.2 159.38,79.33 X4.1
N$45
  Top 1.016: K7_B2.NO 146.3,70.23 144.15,72.39 144.15,79.33 X5.1
N$46
  Top 1.016: K6_B2.NO 128.52,78.95 X6.1
N$47  (via drill 0.5)
  Top 0.254: RN2.2 101.96,21.57 101.73,21.34 101.73,20.07 101.35,19.69 v100.33,19.69
  Top 0.406: IC4.5 104.01,21.08 103.5,21.59 102.55,21.59 RN2.2
  Bottom 0.254: v100.33,19.69 100.97,19.05 100.97,14.99 100.33,14.35 U$18.B1
N$48  (via drill 0.5)
  Top 0.254: v100.97,24.77 101.73,24 101.73,22.61 101.98,22.35 102.51,22.35 RN2.3
  Top 0.406: IC4.4 102.55,22.35 RN2.3
  Bottom 0.406: U$18.B2 101.35,11.81 101.6,12.07 101.6,23.5 100.97,24.13 v100.97,24.77
N$49  (via drill 0.5)
  Top 0.406: IC4.3 102.98,23.62 RN2.4 102.49,23.21 v102.49,24.77
  Bottom 0.406: U$18.B3 102.23,9.27 102.49,9.53 v102.49,24.77
N$50
  Top 0.305: RN5.7 112.5,17.89 113.03,18.41 115.15,18.41 IC4.12 116.91,18.48 118.11,19.69 119.18,19.69 IC5.6
N$51
  Top 0.305: RN5.6 113.3,16.78 113.67,17.14 115.15,17.14 IC4.11 116.91,17.21 118.11,18.41 119.18,18.41 IC5.7
N$52
  Top 0.254: 115.15,15.88 IC4.10
  Top 0.305: RN5.5 114.1,14.83 IC4.10 116.91,15.94 118.11,17.14 119.18,17.14 IC5.8
N$53
  Top 0.406: RN3.1 134.78,13.5 133.99,12.7 120.4,12.7 119.89,12.19 119.89,9.54 R1.C
N$54
  Top 0.406: RN3.2 135.66,18.65 135.89,18.41 135.89,13.34 134.62,12.07 125.98,12.07 125.6,11.68 125.6,9.54 R2.C
N$55
  Top 0.406: RN3.3 136.12,19.45 136.53,19.05 136.53,12.7 135.25,11.43 131.95,11.43 131.32,10.79 131.32,9.54 R3.C
N$56
  Top 0.406: RN3.4 136.59,20.25 137.16,19.69 137.16,10.29 137.03,10.16 137.03,9.54 R4.C
N$57
  Top 0.406: RN4.8 138.5,25.33 139.7,24.13 139.7,14.61 140.97,13.34 159.38,13.34 160.02,12.7 160.02,9.64 R8.C
N$76
  Top 2.54: 74.95,79.35 74.95,76.18 79.38,71.75 79.38,66.55 79.63,66.29
N$77
  Top 2.54: 64.79,79.35 64.79,74.27 67.31,71.75 67.31,66.67 67.69,66.29
N$79
  Top 2.54: 59.71,79.35 59.71,71.73 61.59,69.85 61.59,66.55 61.85,66.29
N$80
  Top 2.54: 49.55,79.35 49.55,66.65 49.91,66.29
N$81
  Top 0.406: RN4.7 138.03,24.53 139.06,23.5 139.06,13.97 140.34,12.7 153.67,12.7 154.31,12.07 154.31,9.64 R7.C
N$82
  Top 0.406: RN4.6 137.56,23.73 138.43,22.86 138.43,13.34 139.7,12.07 147.96,12.07 148.34,11.68 148.34,9.66 R6.C
N$83
  Top 0.406: RN4.5 137.09,22.93 137.79,22.23 137.79,12.7 139.06,11.43 142.24,11.43 142.88,10.79 142.88,9.64 R5.C
N$85
  Top 2.54: 44.47,79.35 44.47,66.7 44.07,66.29
N$86
  Top 2.54: 34.31,79.35 34.31,72.41 32.38,70.49 32.38,66.55 32.13,66.29
N$88
  Top 2.54: 29.23,79.35 29.23,73.68 26.67,71.12 26.67,66.67 26.29,66.29
N$89
  Top 0.305: RN5.8 111.7,18.99 112.39,19.69 115.15,19.69 IC4.13 116.91,19.75 118.11,20.96 119.18,20.96 IC5.5
N$90
  Top 2.54: 19.07,79.35 19.07,75.59 14.61,71.12 14.61,66.55 14.35,66.29
N$93
  Top 0.305: RN6.6 109.62,15.01 110.49,15.88 110.49,20.32 112.39,22.23 115.15,22.23 IC4.15 116.91,22.29 118.11,23.5 119.18,23.5 IC5.3
N$94
  Top 0.305: RN6.8 108.02,15.95 109.22,17.14 109.22,21.59 112.39,24.77 115.12,24.77 IC4.17 116.94,24.86 118.11,26.04 119.18,26.04 IC5.1
N$95
  Bottom 2.54: 14.35,66.29 14.35,70.87 19.05,75.56 19.05,79.33 19.07,79.35
N$96
  Bottom 2.54: 26.29,66.29 26.29,70.1 29.21,73.03 29.21,79.33 29.23,79.35
N$97
  Bottom 2.54: 44.07,66.29 44.07,68.83 44.45,69.22 44.45,79.33 44.47,79.35
N$98
  Bottom 2.54: 61.85,66.29 61.85,69.6 59.69,71.75 59.69,79.33 59.71,79.35
N$99
  Bottom 2.54: 32.13,66.29 32.13,69.6 34.29,71.75 34.29,79.33 34.31,79.35
N$101
  Bottom 2.54: 49.91,66.29 49.91,68.83 49.53,69.22 49.53,78.06 49.55,79.35
N$102
  Top 2.54: 49.53,68.58 49.53,79.38 50.16,79.38 50.16,68.58 | 49.53,68.58 50.16,68.58 | 50.16,68.58 50.16,67.94 | 50.16,67.94 50.16,66.04 49.53,66.04 49.53,66.67 | 49.53,66.67 49.53,67.94 | 49.53,68.58 49.53,67.94 | 49.53,67.94 50.16,67.94 | 49.53,66.67 50.8,66.67 | 50.8,66.67 50.8,79.38 48.26,79.38 48.26,65.41 50.8,65.41 50.8,66.67
N$103
  Bottom 2.54: 54.61,79.33 54.63,79.35
N$106
  Top 2.54: 59.05,72.39 59.05,79.38 60.33,79.38 60.33,73.03 62.87,70.49 62.87,65.41 60.96,65.41 60.96,69.85 | 59.05,72.39 60.96,70.49 60.96,69.85 | 59.05,72.39 59.05,71.75 60.96,69.85
N$107
  Top 2.54: 66.67,65.41 66.67,71.12 64.14,73.66 64.14,79.38 65.41,79.38 65.41,74.29 68.58,71.12 68.58,65.41 66.67,65.41
N$109
  Top 2.54: 74.3,79.38 74.3,76.2 78.74,71.75 78.74,65.41 80.64,65.41 80.64,71.75 75.56,76.84 75.56,79.38 74.3,79.38
N$110
  Top 2.54: 45.09,79.38 45.09,65.41 43.18,65.41 43.18,79.38 45.09,79.38
N$112
  Top 2.54: 34.92,79.38 34.92,72.39 33.66,71.12 33.66,65.41 31.11,65.41 31.11,70.49 33.66,73.03 33.66,79.38 34.92,79.38
N$113
  Top 2.54: 29.21,79.38 29.84,79.38 29.84,73.66 27.3,71.12 27.3,65.41 25.4,65.41 25.4,70.49 28.57,73.66 | 29.21,74.29 29.21,79.38 | 29.21,79.38 28.57,79.38 28.57,73.03
N$115
  Top 2.54: 19.68,79.38 19.68,75.56 15.24,71.12 15.24,65.41 13.34,65.41 13.34,70.49 18.41,75.56 18.41,79.38 19.68,79.38
N$116
  Bottom 2.54: 19.05,79.38 18.41,79.38 18.41,75.56 13.34,70.49 13.34,65.41 15.24,65.41 15.24,71.12 19.68,75.56 19.68,79.38
N$118
  Bottom 2.54: 28.57,79.38 28.57,73.66 25.4,70.49 25.4,65.41 27.3,65.41 27.3,71.12 29.84,73.66 29.84,79.38 28.57,79.38
N$119
  Bottom 2.54: 33.66,79.38 33.66,73.03 31.11,70.49 31.11,65.41 33.66,65.41 33.66,71.12 34.92,72.39 34.92,79.38 33.66,79.38
N$121
  Bottom 2.54: 45.09,79.38 43.18,79.38 43.18,65.41 45.09,65.41 45.09,79.38
N$122
  Bottom 2.54: 48.26,79.38 48.26,65.41 50.8,65.41 50.8,79.38 48.26,79.38
N$124
  Bottom 2.54: 59.05,79.38 59.05,71.75 60.96,69.85 60.96,65.41 62.87,65.41 62.87,70.49 60.33,73.03 60.33,79.38 59.05,79.38
N$125
  Bottom 2.54: 67.69,66.29 67.69,70.1 66.67,71.12 | 66.67,71.12 64.77,73.03 | 64.77,73.03 64.77,79.33 64.79,79.35 | 64.77,73.03 64.14,73.66 64.14,79.38 65.41,79.38 65.41,74.29 68.58,71.12 68.58,65.41 66.67,65.41 66.67,71.12
N$127
  Bottom 2.54: 79.63,66.29 79.63,70.87 78.74,71.75 | 78.74,71.75 74.93,75.56 | 74.93,75.56 74.93,79.33 74.95,79.35 | 74.93,75.56 74.3,76.2 74.3,79.38 75.56,79.38 75.56,76.84 80.64,71.75 80.64,65.41 78.74,65.41 78.74,71.75
N$137
  Top 1.016: K7_B2.NC 134.37,78.99 X5.3
N$138
  Top 1.016: ACS2.4 140.97,51.44 K7_B2.COM 141.6,50.8 | ACS2.3 142.24,50.16 141.6,50.8 | 141.6,50.8 141.6,47.62
N$139
  Top 1.016: K6_B2.NC 116.59,70.87 118.75,73.03 118.75,79.33 X6.3
N$140
  Top 1.016: ACS3.4 123.19,51.44 K6_B2.COM 124.46,50.16 ACS3.3
N$141
  Top 1.016: K5_B2.NC 98.81,71.5 103.5,76.2 103.5,79.33 X7.3
N$142
  Top 1.016: 55.88,67.94 55.88,57.15
N$143
  Top 1.016: K5_B2.NO 110.74,70.74 113.67,73.66 113.67,79.33 X7.1
N$144
  Top 1.016: K4_B2.NO 79.63,71.5 74.93,76.2 74.93,79.33 X8.1
N$145
  Top 1.016: K4_B2.NC 67.69,70.74 64.77,73.66 64.77,79.33 X8.3
N$146
  Top 1.016: ACS5.4 74.3,51.44 K4_B2.COM 74.3,52.07 75.56,50.8 ACS5.3
N$147
  Top 1.016: K3_B2.NO 61.85,70.23 59.69,72.39 59.69,79.33 X9.1
N$148
  Top 1.016: K3_B2.NC 49.91,78.99 X9.3
N$149
  Top 1.016: ACS6.4 56.52,51.44 K3_B2.COM 57.78,50.16 ACS6.3
N$150
  Top 1.016: K2_B2.NO 44.07,78.95 X10.1
N$151
  Top 1.016: K2_B2.NC 32.13,70.87 34.29,73.03 34.29,79.33 X10.3
N$152
  Top 1.016: ACS7.4 38.73,51.44 K2_B2.COM 38.1,52.7 40.01,50.8 ACS7.3
N$153
  Top 1.016: K1_B2.NO 26.29,70.74 29.21,73.66 29.21,79.33 X11.1
N$154
  Top 1.016: K1_B2.NC 14.35,70.87 19.05,75.56 19.05,79.33 X11.3
N$155
  Top 1.016: ACS8.4 20.95,51.44 K1_B2.COM 22.23,50.16 ACS8.3
N$156
  Top 1.016: 57.15,50.16 57.15,47.62
N$157
  Top 1.016: 59.69,52.7 59.69,47.62
N$158
  Top 1.016: 74.93,50.8 74.93,47.62
N$159
  Top 1.016: 77.47,52.7 77.47,49.53 77.47,48.26 77.47,47.62
N$161
  Top 1.016: 70.48,74.93 70.48,76.84 69.85,77.47 69.22,76.84 69.85,76.2 69.85,75.56
N$162
  Top 1.016: 106.05,50.16 106.05,47.62
N$163
  Top 1.016: 108.58,52.7 108.58,47.62
N$164
  Top 1.016: 106.68,54.61 106.68,72.39 109.22,74.93 109.22,77.47 108.58,78.1 107.95,77.47 | 107.95,77.47 107.31,76.84 107.31,74.29 108.58,75.56 108.58,76.84 107.95,77.47 | 107.95,77.47 107.95,74.29 104.14,70.49 104.14,57.79 106.05,55.88 106.05,56.52 106.05,71.12 | 106.05,71.75 106.05,71.12 | 106.05,71.12 104.78,69.85 104.78,58.42 105.41,57.79 105.41,69.85
  Top 1.27: 106.05,55.24 106.05,56.52
N$165
  Top 1.016: 123.83,50.16 123.83,47.62
N$166
  Top 1.016: 126.36,52.7 126.36,47.62 | ACS3.2 125.73,52.7 121.28,57.15 121.28,71.12 121.92,71.75 121.92,77.42 X6.2 125.09,78.1 125.09,55.88 125.09,54.61 127,52.7 ACS3.1
  Top 1.27: 126.36,52.7 126.36,54.61 | 126.36,54.61 125.09,55.88 | 124.46,55.24 125.09,54.61 | 126.36,54.61 126.36,57.15 125.73,57.79 125.73,55.88
N$167
  Top 1.016: 124.46,54.61 122.56,56.52 | 122.56,56.52 121.92,57.15 121.92,70.49 123.19,71.75 123.19,78.74 123.83,79.38 123.83,71.12 | 123.83,71.12 123.83,56.52 124.46,55.88 124.46,78.1 | 122.56,77.47 122.56,56.52 | 122.56,56.52 123.19,57.15 123.19,70.49 123.83,71.12
N$168
  Top 1.016: 144.15,52.7 144.15,47.62
N$170
  Top 1.016: 141.6,68.58 140.97,68.58 139.06,70.49 139.06,77.47 139.7,77.47 | 142.24,54.61 138.43,58.42 138.43,77.47 139.06,78.1 139.7,77.47 | 139.7,77.47 140.34,76.84 140.34,57.15 140.97,56.52 | 140.97,56.52 142.24,55.24 142.24,68.58 140.97,69.85 140.97,56.52 | 140.97,56.52 141.6,57.15 141.6,67.94 | 139.7,77.47 139.7,58.42 | 139.7,57.79 139.7,58.42 | 139.7,58.42 139.06,59.05 139.06,69.85
N$171
  Top 1.016: 159.38,50.16 159.38,47.62
N$172
  Top 1.016: 161.93,52.7 161.93,47.62
N$173
  Top 1.016: 155.57,74.93 155.57,77.47 154.31,78.74 153.67,78.1 153.03,78.1 153.03,76.2 156.21,73.03 156.21,58.42 160.02,54.61 160.02,55.24 | 155.57,74.93 155.57,74.29 160.02,69.85 160.02,55.88 | 155.57,74.93 153.67,76.84 153.67,77.47 154.31,78.1 154.94,77.47 154.94,76.84 | 154.94,76.2 154.94,76.84 | 154.94,76.84 154.31,77.47
N$174
  Top 1.016: 159.38,55.88 159.38,69.85 156.84,72.39 156.84,58.42 157.48,57.79 | 158.12,57.15 158.75,56.52 158.75,69.85 157.48,71.12 157.48,57.79 | 157.48,57.79 158.12,57.15 | 158.12,57.15 158.12,69.85
N$305
  Top 2.54: 149.25,79.35 149.25,73.64 151.76,71.12 151.76,66.67 152.15,66.29
N$306
  Top 2.54: 159.41,79.35 159.41,76.18 163.83,71.75 163.83,66.55 164.08,66.29
N$307
  Top 2.54: 144.17,79.35 144.17,72.37 146.05,70.49 146.05,66.55 146.3,66.29
N$308
  Top 2.54: 128.93,79.35 128.93,66.7 128.52,66.29
N$309
  Top 2.54: 134.01,79.35 134.01,66.65 134.37,66.29
N$311
  Top 2.54: 118.77,79.35 118.77,72.41 116.84,70.49 116.84,66.55 116.59,66.29
N$313
  Top 2.54: 103.53,79.35 103.53,75.59 98.42,70.49 98.42,66.67 98.81,66.29
N$315
  Top 2.54: 113.69,79.35 113.69,73.68 110.49,70.49 110.49,66.55 110.74,66.29
N$360
  Top 2.54: 113.69,79.35 113.69,73.68 111.12,71.12 111.12,66.67 110.74,66.29
N$361
  Top 2.54: 103.53,79.35 103.53,75.59 99.06,71.12 99.06,66.55 98.81,66.29
N$363
  Top 2.54: 128.93,79.35 128.93,66.7 128.52,66.29
N$364
  Top 2.54: 118.77,79.35 118.77,72.41 116.84,70.49 116.84,66.55 116.59,66.29
N$366
  Top 2.54: 144.17,79.35 144.17,71.73 146.05,69.85 146.05,66.55 146.3,66.29
N$367
  Top 2.54: 134.01,79.35 134.01,66.65 134.37,66.29
N$369
  Top 2.54: 159.41,79.35 159.41,76.18 163.83,71.75 163.83,66.55 164.08,66.29
N$370
  Top 2.54: 149.25,79.35 149.25,74.27 152.4,71.12 152.4,66.55 152.15,66.29
N$373
  Bottom 2.54: 98.81,66.29 98.81,70.87 103.5,75.56 103.5,79.33 103.53,79.35
N$374
  Bottom 2.54: 110.74,66.29 110.74,70.1 113.67,73.03 113.67,79.33 113.69,79.35
N$375
  Bottom 2.54: 128.52,66.29 128.52,68.83 128.91,69.22 128.91,79.33 128.93,79.35
N$376
  Bottom 2.54: 146.3,66.29 146.3,69.6 144.15,71.75 144.15,79.33 144.17,79.35
N$377
  Bottom 2.54: 116.59,66.29 116.59,69.6 118.75,71.75 118.75,79.33 118.77,79.35
N$379
  Bottom 2.54: 134.37,66.29 134.37,68.83 133.99,69.22 133.99,78.06 134.01,79.35
N$380
  Top 2.54: 133.99,68.58 133.99,79.38 134.62,79.38 134.62,68.58 | 133.99,68.58 134.62,68.58 | 134.62,68.58 134.62,67.94 | 134.62,67.94 134.62,66.04 133.99,66.04 133.99,66.67 | 133.99,66.67 133.99,67.94 | 133.99,68.58 133.99,67.94 | 133.99,67.94 134.62,67.94 | 133.99,66.67 135.25,66.67 | 135.25,66.67 135.25,79.38 132.72,79.38 132.72,65.41 135.25,65.41 135.25,66.67
N$383
  Top 2.54: 143.51,79.38 143.51,71.75 145.41,69.85 145.41,65.41 147.32,65.41 147.32,70.49 144.78,73.03 144.78,79.38 143.51,79.38
N$384
  Top 2.54: 151.13,65.41 151.13,71.12 148.59,73.66 148.59,79.38 149.86,79.38 149.86,74.29 153.03,71.12 153.03,65.41 151.13,65.41
N$386
  Top 2.54: 158.75,79.38 158.75,76.2 163.19,71.75 163.19,65.41 165.1,65.41 165.1,71.75 160.02,76.84 160.02,79.38 158.75,79.38
N$387
  Top 2.54: 129.54,79.38 129.54,65.41 127.64,65.41 127.64,79.38 129.54,79.38
N$389
  Top 2.54: 119.38,79.38 119.38,72.39 118.11,71.12 118.11,65.41 115.57,65.41 115.57,70.49 118.11,73.03 118.11,79.38 119.38,79.38
N$390
  Top 2.54: 113.67,79.38 114.3,79.38 114.3,73.66 111.76,71.12 111.76,65.41 109.86,65.41 109.86,70.49 113.03,73.66 | 113.67,74.29 113.67,79.38 | 113.67,79.38 113.03,79.38 113.03,73.03
N$392
  Top 2.54: 104.14,79.38 104.14,75.56 99.69,71.12 99.69,65.41 97.79,65.41 97.79,70.49 102.87,75.56 102.87,79.38 104.14,79.38
N$393
  Bottom 2.54: 103.5,79.38 102.87,79.38 102.87,75.56 97.79,70.49 97.79,65.41 99.69,65.41 99.69,71.12 104.14,75.56 104.14,79.38
N$395
  Bottom 2.54: 113.03,79.38 113.03,73.66 109.86,70.49 109.86,65.41 111.76,65.41 111.76,71.12 114.3,73.66 114.3,79.38 113.03,79.38
N$396
  Bottom 2.54: 118.11,79.38 118.11,73.03 115.57,70.49 115.57,65.41 118.11,65.41 118.11,71.12 119.38,72.39 119.38,79.38 118.11,79.38
N$398
  Bottom 2.54: 129.54,79.38 127.64,79.38 127.64,65.41 129.54,65.41 129.54,79.38
N$399
  Bottom 2.54: 132.72,79.38 132.72,65.41 135.25,65.41 135.25,79.38 132.72,79.38
N$401
  Bottom 2.54: 143.51,79.38 143.51,71.75 145.41,69.85 145.41,65.41 147.32,65.41 147.32,70.49 144.78,73.03 144.78,79.38 143.51,79.38
N$402
  Bottom 2.54: 152.15,66.29 152.15,70.1 151.13,71.12 | 151.13,71.12 149.22,73.03 | 149.22,73.03 149.22,79.33 149.25,79.35 | 149.22,73.03 148.59,73.66 148.59,79.38 149.86,79.38 149.86,74.29 153.03,71.12 153.03,65.41 151.13,65.41 151.13,71.12
N$404
  Bottom 2.54: 164.08,66.29 164.08,70.87 163.19,71.75 | 163.19,71.75 159.38,75.56 | 159.38,75.56 159.38,79.33 159.41,79.35 | 159.38,75.56 158.75,76.2 158.75,79.38 160.02,79.38 160.02,76.84 165.1,71.75 165.1,65.41 163.19,65.41 163.19,71.75
OC_R1  (via drill 0.5)
  Top 0.305: IC5.11 131.32,17.27 131.95,17.91 133.13,17.91 RN3.8
  Top 0.406: v127,17.14 128.98,17.14 IC5.11
  Bottom 0.406: K8_B2.C1 165.61,54.1 167,52.7 167,18.41 165.74,17.14 v127,17.14
OC_R2  (via drill 0.5)
  Top 0.305: IC5.12 131.44,18.54 131.57,18.67 133.17,18.67 RN3.7
  Top 0.406: v127,18.41 128.98,18.41 IC5.12
  Bottom 0.406: K7_B2.C1 147.83,54.1 149.22,52.7 149.22,19.69 147.96,18.41 v127,18.41
OC_R3  (via drill 0.5)
  Top 0.305: IC5.13 131.32,19.81 131.7,19.43 133.17,19.43 RN3.6
  Top 0.406: v127,19.69 128.98,19.69 IC5.13
  Bottom 0.406: K6_B2.C1 130.05,54.1 131.44,52.7 131.44,21.08 130.18,19.81 127.13,19.81 v127,19.69
OC_R4  (via drill 0.5)
  Top 0.305: IC5.14 131.32,21.08 132.08,20.32 133.12,20.32 RN3.5
  Top 0.406: v127,20.96 128.98,20.96 IC5.14
  Bottom 0.406: K5_B2.C1 112.27,54.1 113.67,52.7 113.67,46.99 115.57,45.09 129.54,45.09 130.18,44.45 130.18,22.15 IC5.14 127.13,21.08 v127,20.96
OC_R5  (via drill 0.5)
  Top 0.305: IC5.15 131.57,22.35 132.08,22.86 133.12,22.86 RN4.4
  Top 0.406: v127,22.23 128.98,22.23 IC5.15
  Bottom 0.406: K4_B2.C1 79.63,50.93 81.03,49.53 95.25,49.53 96.52,48.26 96.52,45.09 97.16,44.45 128.91,44.45 129.54,43.81 129.54,22.78 IC5.15 127.13,22.35 v127,22.23
OC_R6  (via drill 0.5)
  Top 0.305: IC5.16 133.08,23.62 RN4.3
  Top 0.406: v127,23.5 128.98,23.5 IC5.16
  Bottom 0.406: K3_B2.C1 64.01,54.1 64.77,53.34 64.77,50.8 66.67,48.9 94.61,48.9 95.89,47.62 95.89,44.45 96.52,43.81 128.27,43.81 128.91,43.18 128.91,24.13 128.27,23.5 v127,23.5
OC_R7  (via drill 0.5)
  Top 0.305: IC5.17 131.32,24.89 131.7,24.51 133.17,24.51 RN4.2
  Top 0.406: v127,24.77 128.98,24.77 IC5.17
  Bottom 0.406: K2_B2.C1 46.23,54.1 46.99,53.34 46.99,50.8 49.53,48.26 93.98,48.26 95.25,46.99 95.25,43.81 95.89,43.18 127.64,43.18 128.27,42.55 128.27,25.4 127.64,24.77 v127,24.77
OC_R8  (via drill 0.5)
  Top 0.305: IC5.18 131.19,26.16 132.08,25.27 133.13,25.27 RN4.1
  Top 0.406: v127,26.04 128.98,26.04 IC5.18
  Bottom 0.406: K1_B2.C1 28.45,54.1 29.21,53.34 29.21,50.8 32.38,47.62 93.34,47.62 94.61,46.35 94.61,43.18 95.25,42.55 126.36,42.55 127,41.91 v127,26.04
REG_5V  (via drill 0.5, 0.9)
  Top 0.254: U$4.B2 U$4.B1 | v70.48,26.16 CA4.1 | 113.03,26.67 108.58,22.23 108.58,20.45 107.95,19.81 | IC3.16 66.41,28.31 v67.31,29.21 | v62.48,28.7 62.48,27.48 IC3.10 62.48,27.43 62.48,26.67 61.85,26.04 60.96,26.04 | RNE.6 RNE.5
  Top 0.305: H1.1 6.19,19.27 4.95,18.03 4.95,15.83 RNB.6
  Top 0.406: IC3.16 70.23,27.46 CA4.1 75.33,27.71 76.2,28.57 76.2,30.48 C1.+ | CB3.2 84.22,29.62 | IC4.18 113.54,26.16 113.03,26.67 v113.03,27.94 113.03,30.12 CB6.2 CA7.2 | 127,7.62 121.92,7.62 121.4,8.14 R1.A 121.4,11.32 v121.28,11.43 | 127,7.62 132.72,7.62 | 132.72,7.62 138.43,7.62 | 138.43,7.62 144.15,7.62 | 144.15,7.62 149.86,7.62 | 149.86,7.62 155.57,7.62 | 155.57,7.62 160.66,7.62 161.29,8.26 161.29,9.41 R8.A | R7.A 155.69,7.74 155.57,7.62 | R6.A 149.97,7.74 149.86,7.62 | R5.A 144.26,7.74 144.15,7.62 | R4.A 138.54,7.74 138.43,7.62 | R3.A 132.83,7.74 132.72,7.62 | R2.A 127.11,7.74 127,7.62 | 107.95,19.81 IC4.6 105.89,19.69 103.5,19.69 102.23,18.41 99.69,18.41 99.06,17.78 99.06,16.51 98.42,15.88 94.61,15.88 93.98,15.24 U$18.A1 U$18.A2 U$18.A3 | RNE.5 45.55,28.74 46.35,27.94 X3.2
  Top 0.762: 83.82,28.57 84.45,27.94 107.95,27.94 108.58,28.57 108.58,29.82
  Top 0.813: 16.13,20.83 9.96,20.83 H1.1 | 16.13,20.83 17.27,20.83 18.41,19.69 20.75,19.69 C13.1 | IC1.4 16.13,19.15 16.13,20.83 | S1.1 57.78,3.81 58.42,4.45 58.42,23.5 60.96,26.04
  Top 1.016: C1.+ 76.83,29.84 78.11,28.57 83.82,28.57 84.45,29.21 84.45,29.87 CB3.2 CA3.2 82.55,33.02 v81.92,33.66 | 108.58,29.82 CA7.2 | v87,46.35 87,50.8 90.55,54.36 90.55,60.45 C10.+ | 46.35,2.16 46.35,1.52 | 46.35,1.52 15.37,1.52 11.3,5.59 11.3,14.35 9.27,16.38 9.27,18.41 H1.1 | 22.05,19.69 22.23,19.69 22.86,20.32 22.86,28.57 v23.5,29.21 | S1.1 53.98,2.41 53.09,1.52 46.35,1.52
  Top 1.27: 20.75,19.69 22.05,19.69
  Top 1.778: X3.2 46.35,2.16
  Bottom 0.254: U$4.B1 76.2,15.24 75.56,15.88 71.12,15.88 70.48,16.51 v70.48,26.16 | v67.31,29.21 62.87,29.21 v62.48,28.7
  Bottom 0.406: v121.28,11.43 114.3,11.43 113.67,12.07 113.67,27.3 v113.03,27.94
  Bottom 1.016: v81.92,33.66 85.72,33.66 87,34.92 v87,46.35
REG_5V_A  (via drill 0.5)
  Top 0.406: ACS1.8 162.56,45.09 | ACS2.8 144.78,45.09 | ACS3.8 127,45.09 | ACS4.8 109.22,45.09
  Top 1.016: C3.2 C5.2 87.55,16.28 U$5.OUT 89.31,19.91 v88.9,20.32 | v89.53,45.09 109.22,45.09 127,45.09 144.78,45.09 162.56,45.09
  Bottom 1.016: v88.9,20.32 88.9,44.45 v89.53,45.09
REG_5V_B  (via drill 0.5)
  Top 0.406: ACS5.8 v78.11,45.09 | ACS6.8 v60.33,45.09 | ACS7.8 42.55,45.09 | ACS8.8 24.77,45.09
  Top 1.016: U$6.OUT 69.47,18.04 67.94,16.51 66.27,16.51 C9.2 C7.2 60.55,16.28 v60.33,16.51 | 24.77,45.09 42.55,45.09 v48.26,45.09 v78.11,45.09
  Bottom 1.143: 58.42,37.47 49.53,37.47
  Bottom 1.27: v60.33,16.51 60.33,35.56 58.42,37.47 | 49.53,37.47 48.26,38.73 v48.26,45.09 | v78.11,45.09 v60.33,45.09
REG_12V  (via drill 0.5)
  Top 0.61: IC1.7 13.46,23.16 | 14.1,22.48 14.15,22.48
  Top 0.813: v18.41,22.48 14.15,22.48 13.46,23.16 | v25.4,22.48 26.04,22.48 26.67,21.84 C12.1 26.67,14.61 27.94,13.34 BRA1.+
  Bottom 0.813: v18.41,22.48 v25.4,22.48
UNREG_12V  (via drill 0.5, 0.9)
  Top 0.406: v132.08,15.24 131.57,15.24 130.81,16 IC5.10
  Top 1.016: BRA4.~@2 BRA4.~@1 BRA3.~@2 BRA3.~@1 v62.87,6.99
  Top 1.27: C11.+ v154.94,15.24 | K1_B2.C2 14.35,34.54 15.24,33.66 v31.11,33.66
  Top 2.54: X2.2 28.87,5.42 24.13,10.16 BRA1.~@1 24.13,15.24 | 24.13,15.24 BRA1.~@2 | U$1.TIP 15.14,13.87 16.51,15.24 24.13,15.24
  Bottom 1.016: v62.87,6.99 62.87,11.43 60.96,13.34 59.05,13.34 58.42,13.97 58.42,33.02 57.78,33.66 v31.11,33.66 | C11.+ 154.94,33.02 152.4,35.56 152.4,53.85 K8_B2.C2 152.15,55.5 150.5,57.15 134.62,57.15 | 134.62,57.15 116.84,57.15 | 116.84,57.15 99.06,57.15 | 99.06,57.15 67.94,57.15 | 67.94,57.15 50.16,57.15 | 50.16,57.15 32.38,57.15 | 32.38,57.15 14.61,57.15 13.97,56.52 13.97,54.48 K1_B2.C2 | K2_B2.C2 32.13,56.9 32.38,57.15 | K3_B2.C2 49.91,56.9 50.16,57.15 | K4_B2.C2 67.69,56.9 67.94,57.15 | K5_B2.C2 98.81,56.9 99.06,57.15 | K6_B2.C2 116.59,56.9 116.84,57.15 | K7_B2.C2 134.37,56.9 134.62,57.15
  Bottom 1.27: v154.94,15.24 v132.08,15.24
  Bottom 1.778: v31.11,33.66 31.11,6.71 X2.2

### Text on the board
tNames: IP- | IP+ | IP- | IP- | IP+ | IP- | IP- | IP+ | IP- | IP- | IP+ | IP- | IP- | IP+ | IP- | IP- | IP+ | IP- | IP- | IP+ | IP- | IP- | IP+ | IP- | NC | COM | NO | NC | COM | NO | NC | COM | NO | NC | COM | NO | NC | COM | NO | NC | COM | NO | NC | COM | NO | NC | COM | NO | 8 | 5 | 4 | 1 | Bank 1 | 8 | 8 | 7 | 7 | 6 | 6 | 5 | 5 | 4 | 4 | 3 | 3 | 2 | 2 | 1 | 1 | 2016 ControlEverything.com | SC | ADS7828 | MCP23008 | I2C OUT | SCCMR8x | REV.A | SCL | SDA | +5V | GND | A1 | A0 | A1 | A1 | A0 | A2 | ADC / Address | Relay Address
